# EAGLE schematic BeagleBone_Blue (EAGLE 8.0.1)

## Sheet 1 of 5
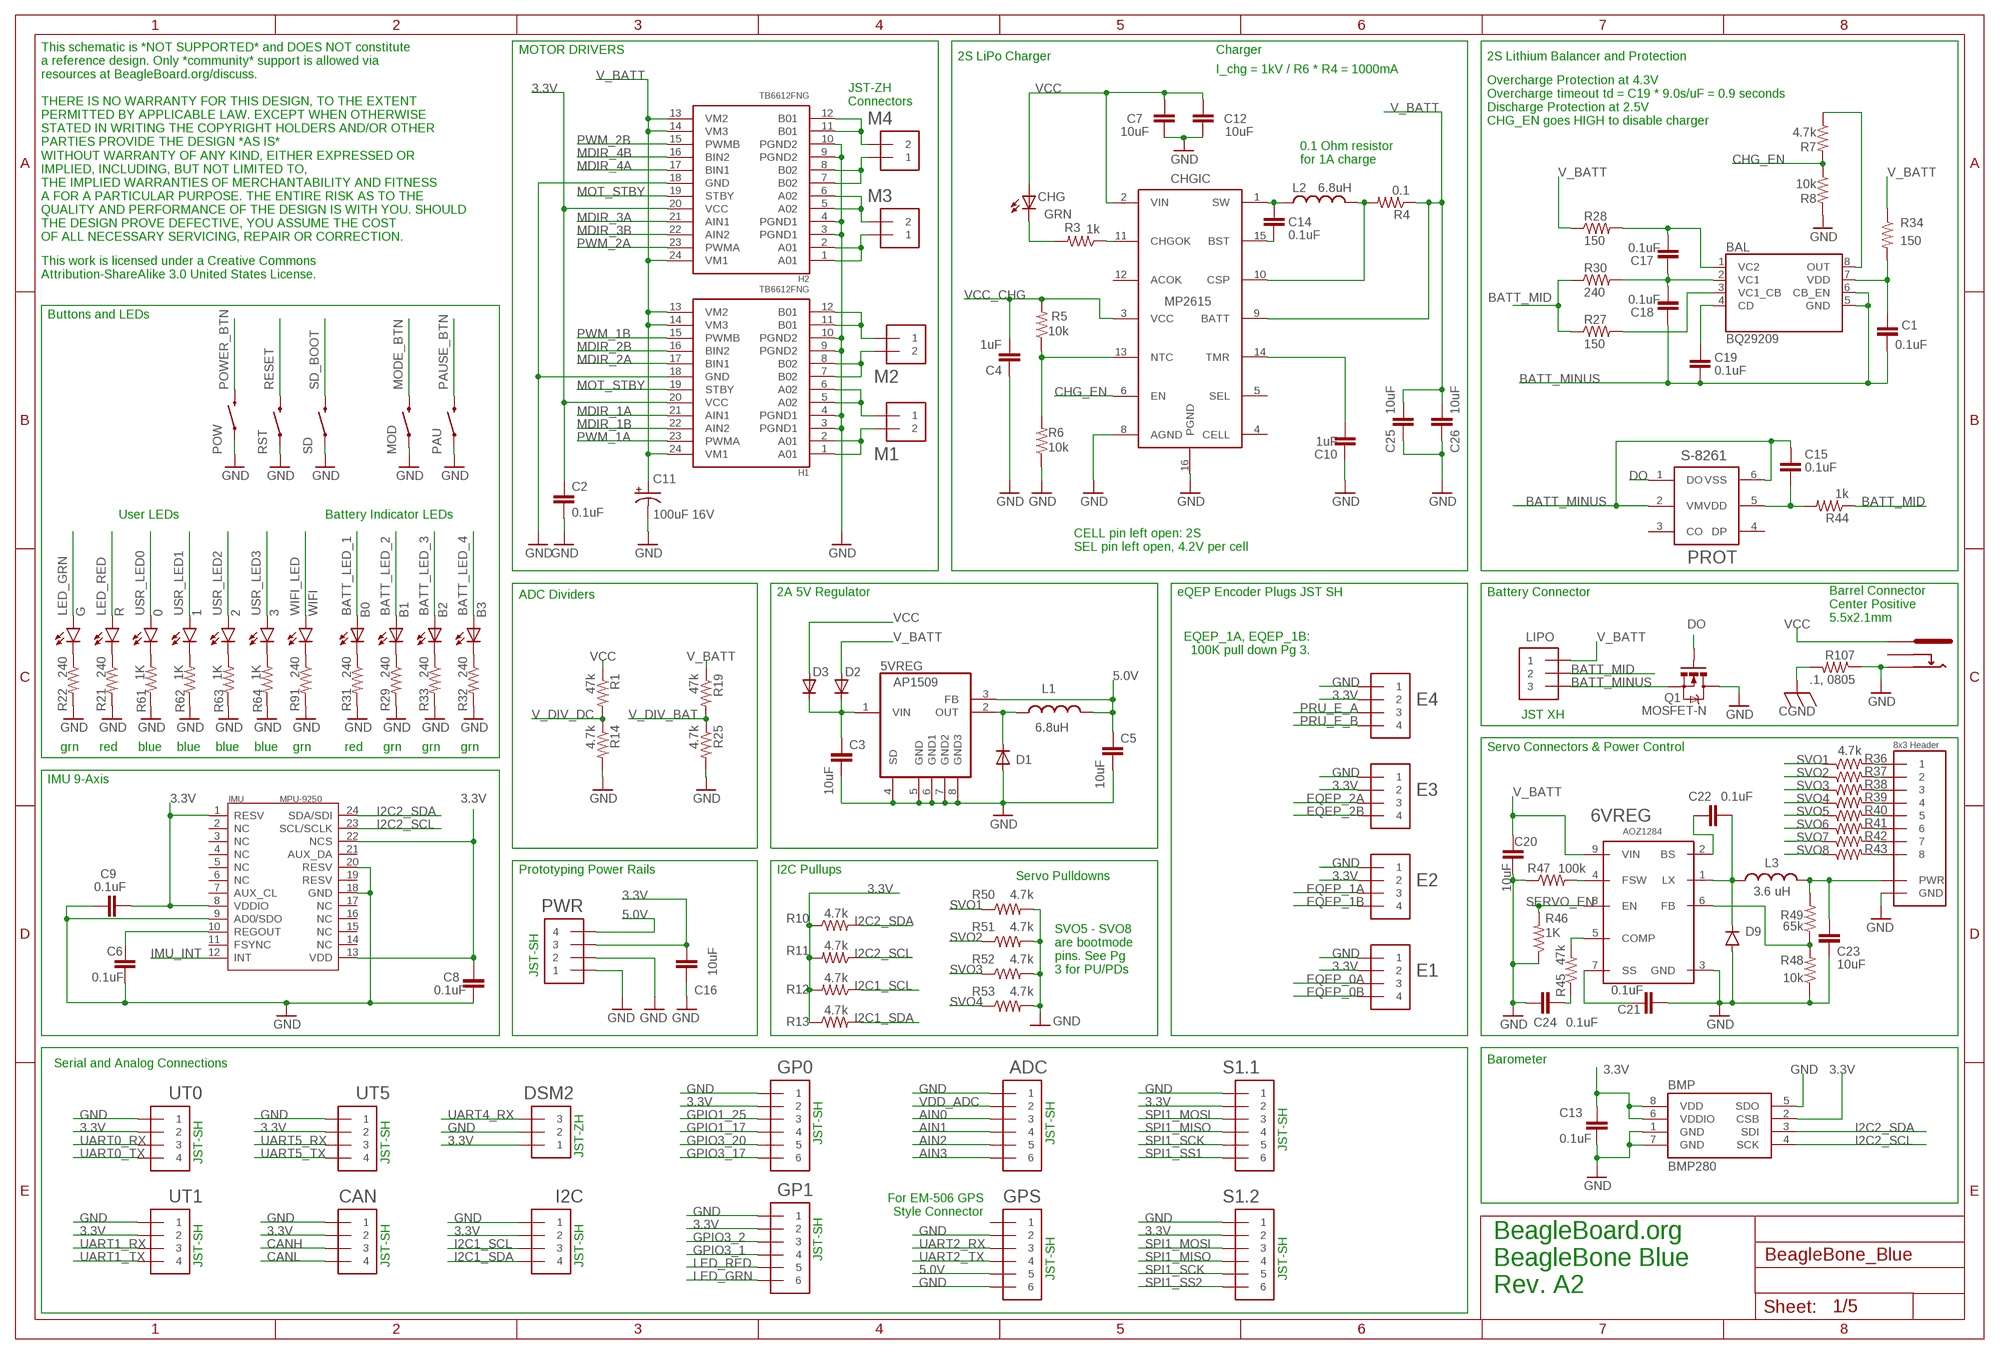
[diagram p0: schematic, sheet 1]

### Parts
0  BLUE  LED0603  [BEAGLEBONE_BLUE_LED-0603]
1  BLUE  LED0603  [BEAGLEBONE_BLUE_LED-0603]
2  BLUE  LED0603  [BEAGLEBONE_BLUE_LED-0603]
3  BLUE  LED0603  [BEAGLEBONE_BLUE_LED-0603]
5VREG  AP1509SOIC-8-TIGHT  [BEAGLEBONE_BLUE_SO08-TIGHT]
6VREG  AOZ1284  [SO08-EXPOSED]
12V  PJ-102B_POWER_CON  [PJ-102B_POWER_CON]
ADC  JST_SH_6  [JST_SH_6]
B0  RED  LED0603  [LED-0603]
B1  GREEN  LED0603  [LED-0603]
B2  GREEN  LED0603  [LED-0603]
B3  GREEN  LED0603  [LED-0603]
BAL  BQ29209  [8-SON_3X3MM]
BMP  BMP280  [BMP280]
C1  0.1uF  CAP0402-CAP  [0402-CAP]
C2  0.1uF  CAP0402-CAP  [0402-CAP]
C3  10uF  CAP0805  [0805]
C4  1uF  CAP0402-CAP  [0402-CAP]
C5  10uF  CAP0805  [0805]
C6  0.1uF  CAP0402-CAP  [0402-CAP]
C7  10uF  CAP0805  [0805]
C8  0.1uF  CAP0402-CAP  [0402-CAP]
C9  0.1uF  CAP0402-CAP  [0402-CAP]
C10  1uF  CAP0402-CAP  [0402-CAP]
C11  100uF 16V  CPOL-USD  [PANASONIC_D]
C12  10uF  CAP0805  [0805]
C13  0.1uF  CAP0402-CAP  [0402-CAP]
C14  0.1uF  CAP0402-CAP  [0402-CAP]
C15  0.1uF  CAP0402-CAP  [0402-CAP]
C16  10uF  CAP0805  [0805]
C17  0.1uF  CAP0402-CAP  [0402-CAP]
C18  0.1uF  CAP0402-CAP  [0402-CAP]
C19  0.1uF  CAP0402-CAP  [0402-CAP]
C20  10uF  CAP0805  [0805]
C21  0.1uF  CAP0402-CAP  [0402-CAP]
C22  0.1uF  CAP0402-CAP  [0402-CAP]
C23  10uF  CAP0805  [0805]
C24  0.1uF  CAP0402-CAP  [0402-CAP]
C25  10uF  CAP0805  [0805]
C26  10uF  CAP0805  [0805]
CAN  JST_SH_4  [JST_SH_4_SMD]
CHG  GRN  LED0603  [LED-0603]
CHGIC  MP2615  [MP2615]
D1  DIODE_SOD-123FL  [ADAFRUIT_SOD-123FL]
D2  DIODE_SOD-123FL  [ADAFRUIT_SOD-123FL]
D3  DIODE_SOD-123FL  [ADAFRUIT_SOD-123FL]
D9  DIODEDO214AA  [DO-214AA]
DSM2  JST_ZH_3  [JST_ZH_3]
E1  JST_SH_4  [JST_SH_4_SMD]
E2  JST_SH_4  [JST_SH_4_SMD]
E3  JST_SH_4  [JST_SH_4_SMD]
E4  JST_SH_4  [JST_SH_4_SMD]
G  GREEN  LED0603  [BEAGLEBONE_BLUE_LED-0603]
GP0  JST_SH_6  [JST_SH_6]
GP1  JST_SH_6  [JST_SH_6]
GPS  JST_SH_6  [JST_SH_6]
H1  TB6612FNG  [SSOP24]
H2  TB6612FNG  [SSOP24]
I2C  JST_SH_4  [JST_SH_4_SMD]
IMU  MPU-9250  [QFN24G-0.4-3X3MM]
J2  STRAWSON_EAGLE_LIB_SERVO_HEADERS_8X  [STRAWSON_EAGLE_LIB_3X8_0.1"_HEADER]
L1  6.8uH  INDUCTORBOURNS_SRN6045  [SRN6045]
L2  6.8uH  INDUCTORBOURNS_SRN6045  [SRN6045]
L3  3.6 uH  INDUCTOR  [8X8MM_INDUCTOR]
LIPO  BATTERY  JST_XH_3-PIN  [JST_XH_3-PIN]
M1  JST_ZH_2  [JST_ZH_2]
M2  JST_ZH_2  [JST_ZH_2]
M3  JST_ZH_2  [JST_ZH_2]
M4  JST_ZH_2  [JST_ZH_2]
MOD  SWITCH-MOMENTARY-2SMD-1101NE  [TACTILE-SWITCH-1101NE]
PAU  SWITCH-MOMENTARY-2SMD-1101NE  [TACTILE-SWITCH-1101NE]
POW  SWITCH-MOMENTARY-2SMD-1101NE  [TACTILE-SWITCH-1101NE]
PROT  S-8261  [SOT-236]
PWR  JST_SH_4  [JST_SH_4_SMD]
Q1  MOSFET-N  MOSFET-NCHANNEL  [SO08-TIGHT]
R  RED  LED0603  [BEAGLEBONE_BLUE_LED-0603]
R1  47k  RESISTOR0402-RES  [0402-RES]
R3  1k  RESISTOR0402-RES  [0402-RES]
R4  0.1  RESISTOR0603  [0603-RES]
R5  10k  RESISTOR0402-RES  [0402-RES]
R6  10k  RESISTOR0402-RES  [0402-RES]
R7  4.7k  RESISTOR0402-RES  [0402-RES]
R8  10k  RESISTOR0402-RES  [0402-RES]
R10  4.7k  RESISTOR0402-RES  [0402-RES]
R11  4.7k  RESISTOR0402-RES  [0402-RES]
R12  4.7k  RESISTOR0402-RES  [0402-RES]
R13  4.7k  RESISTOR0402-RES  [0402-RES]
R14  4.7k  RESISTOR0402-RES  [0402-RES]
R19  47k  RESISTOR0402-RES  [0402-RES]
R21  240  RESISTOR0402-RES  [0402-RES]
R22  240  RESISTOR0402-RES  [0402-RES]
R25  4.7k  RESISTOR0402-RES  [0402-RES]
R27  150  RESISTOR0402-RES  [0402-RES]
R28  150  RESISTOR0402-RES  [0402-RES]
R29  240  RESISTOR0402-RES  [0402-RES]
R30  240  RESISTOR0402-RES  [0402-RES]
R31  240  RESISTOR0402-RES  [0402-RES]
R32  240  RESISTOR0402-RES  [0402-RES]
R33  240  RESISTOR0402-RES  [0402-RES]
R34  150  RESISTOR0402-RES  [0402-RES]
R36  4.7k  RESISTOR0402-RES  [0402-RES]
R37  4.7k  RESISTOR0402-RES  [0402-RES]
R38  4.7k  RESISTOR0402-RES  [0402-RES]
R39  4.7k  RESISTOR0402-RES  [0402-RES]
R40  4.7k  RESISTOR0402-RES  [0402-RES]
R41  4.7k  RESISTOR0402-RES  [0402-RES]
R42  4.7k  RESISTOR0402-RES  [0402-RES]
R43  4.7k  RESISTOR0402-RES  [0402-RES]
R44  1k  RESISTOR0402-RES  [0402-RES]
R45  47k  RESISTOR0402-RES  [0402-RES]
R46  1K  RESISTOR0402-RES  [0402-RES]
R47  100k  RESISTOR0402-RES  [0402-RES]
R48  10k  RESISTOR0402-RES  [0402-RES]
R49  65k  RESISTOR0402-RES  [0402-RES]
R50  4.7k  RESISTOR0402-RES  [0402-RES]
R51  4.7k  RESISTOR0402-RES  [0402-RES]
R52  4.7k  RESISTOR0402-RES  [0402-RES]
R53  4.7k  RESISTOR0402-RES  [0402-RES]
R61  1K  RESISTOR0402-RES  [0402-RES]
R62  1K  RESISTOR0402-RES  [0402-RES]
R63  1K  RESISTOR0402-RES  [0402-RES]
R64  1K  RESISTOR0402-RES  [0402-RES]
R91  240  RESISTOR0402-RES  [0402-RES]
R107  .1, 0805  R-US_R0805  [R0805]
RST  SWITCH-MOMENTARY-2SMD-1101NE  [TACTILE-SWITCH-1101NE]
S1.1  JST_SH_6  [JST_SH_6]
S1.2  JST_SH_6  [JST_SH_6]
SD  SWITCH-MOMENTARY-2SMD-1101NE  [TACTILE-SWITCH-1101NE]
UT0  JST_SH_4  [JST_SH_4_SMD]
UT1  JST_SH_4  [JST_SH_4_SMD]
UT5  JST_SH_4  [JST_SH_4_SMD]
WIFI  GREEN  LED0603  [BEAGLEBONE_BLUE_LED-0603]

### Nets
3.3V: BMP.2(CSB) BMP.6(VDDIO) BMP.8(VDD) C2.2 C8.1 C9.2 C13.1 C16.1 CAN.2 DSM2.P$1 E1.2 E2.2 E3.2 E4.2 GP0.2 GP1.2 H1.20(VCC) H2.20(VCC) I2C.2 IMU.1(RESV) IMU.8(VDDIO) IMU.13(VDD) IMU.22(NCS) PWR.3 R10.1 R11.2 R12.2 R13.1 S1.1.2 S1.2.2 UT0.2 UT1.2 UT5.2 ; also sheet 2,3,5
5.0V [power]: 5VREG.3(FB) C5.1 GPS.5 L1.2 PWR.4 ; also sheet 2,3
AIN0: ADC.3 ; also sheet 3
AIN1: ADC.4 ; also sheet 3
AIN2: ADC.5 ; also sheet 3
AIN3: ADC.6 ; also sheet 3
BATT_LED_1: B0.A ; also sheet 2
BATT_LED_2: B1.A ; also sheet 3
BATT_LED_3: B2.A ; also sheet 2
BATT_LED_4: B3.A ; also sheet 2
BATT_MID: LIPO.P$2 R27.1 R30.1 R44.1
BATT_MINUS: BAL.5(GND) BAL.6(CB_EN) C1.2 C15.1 C18.1 C19.2 LIPO.P$3 PROT.2(VM) PROT.6(VSS) Q1.1(S) Q1.2(S) Q1.3(S)
CANH: CAN.3 ; also sheet 2
CANL: CAN.4 ; also sheet 2
CGND: R107.2 ; also sheet 2,3,4
CHG_EN: CHGIC.6(EN) R7.2 R8.1
CO: BAL.8(OUT) R7.1
DO: PROT.1(DO) Q1.4(G)
EQEP_0A: E1.3 ; also sheet 2
EQEP_0B: E1.4 ; also sheet 2
EQEP_1A: E2.3 ; also sheet 3
EQEP_1B: E2.4 ; also sheet 3
EQEP_2A: E3.3 ; also sheet 2
EQEP_2B: E3.4 ; also sheet 2
GND [ground]: 5VREG.4(SD) 5VREG.5(GND) 5VREG.6(GND1) 5VREG.7(GND2) 5VREG.8(GND3) 6VREG.3(GND) 12V.OUT ADC.1 BMP.1(GND) BMP.5(SDO) BMP.7(GND) C2.1 C3.2 C4.1 C5.2 C6.2 C7.2 C8.2 C9.1 C10.1 C11.- C12.2 C13.2 C16.2 C20.1 C21.1 C23.1 C24.1 C25.2 C26.2 CAN.1 CHGIC.8(AGND) CHGIC.16(PGND) D1.A D9.A DSM2.P$2 E1.1 E2.1 E3.1 E4.1 GP0.1 GP1.1 GPS.2 GPS.6 H1.3(PGND1) H1.4(PGND1) H1.9(PGND2) H1.10(PGND2) H1.18(GND) H2.3(PGND1) H2.4(PGND1) H2.9(PGND2) H2.10(PGND2) H2.18(GND) I2C.1 IMU.9(AD0/SDO) IMU.18(GND) IMU.20(RESV) J2.P$13(GND) J2.P$14(GND) J2.P$15(GND) J2.P$16(GND) J2.P$17(GND) J2.P$18(GND) J2.P$23(GND) J2.P$24(GND) MOD.1 PAU.1 POW.1 PWR.1 PWR.2 Q1.5(D) Q1.6(D) Q1.7(D) Q1.8(D) R6.1 R8.2 R14.2 R21.2 R22.2 R25.2 R29.2 R31.2 R32.2 R33.2 R46.1 R47.1 R48.1 R50.2 R51.2 R52.2 R53.2 R61.1 R62.1 R63.1 R64.1 R91.2 R107.1 RST.1 S1.1.1 S1.2.1 SD.1 UT0.1 UT1.1 UT5.1 ; also sheet 2,3,4,5
GPIO1_17: GP0.4 ; also sheet 2
GPIO1_25: GP0.3 ; also sheet 3
GPIO3_1: GP1.4 ; also sheet 3
GPIO3_2: GP1.3 ; also sheet 3
GPIO3_17: GP0.6 ; also sheet 2
GPIO3_20: GP0.5 ; also sheet 2
I2C1_SCL: I2C.3 R12.1 ; also sheet 2
I2C1_SDA: I2C.4 R13.2 ; also sheet 2
I2C2_SCL: BMP.4(SCK) IMU.23(SCL/SCLK) R11.1 ; also sheet 2
I2C2_SDA: BMP.3(SDI) IMU.24(SDA/SDI) R10.2 ; also sheet 2
IMU_INT: IMU.12(INT) ; also sheet 2
L3: B2.C R33.1
L4: B3.C R32.1
LED_GRN: G.A GP1.6 ; also sheet 2
LED_RED: GP1.5 R.A ; also sheet 2
MDIR_1A: H1.21(AIN1) ; also sheet 2
MDIR_1B: H1.22(AIN2) ; also sheet 2
MDIR_2A: H1.17(BIN1) ; also sheet 2
MDIR_2B: H1.16(BIN2) ; also sheet 3
MDIR_3A: H2.21(AIN1) ; also sheet 3
MDIR_3B: H2.22(AIN2) ; also sheet 3
MDIR_4A: H2.17(BIN1) ; also sheet 3
MDIR_4B: H2.16(BIN2) ; also sheet 3
MODE_BTN: MOD.2 ; also sheet 2
MOT1A: H1.1(A01) H1.2(A01) M1.P$2
MOT1B: H1.5(A02) H1.6(A02) M1.P$1
MOT2A: H1.11(B01) H1.12(B01) M2.P$1
MOT2B: H1.7(B02) H1.8(B02) M2.P$2
MOT3A: H2.1(A01) H2.2(A01) M3.P$1
MOT3B: H2.5(A02) H2.6(A02) M3.P$2
MOT4A: H2.11(B01) H2.12(B01) M4.P$2
MOT4B: H2.7(B02) H2.8(B02) M4.P$1
MOT_STBY: H1.19(STBY) H2.19(STBY) ; also sheet 2
N$1: J2.P$1 R36.2
N$3: G.C R22.1
N$4: BAL.2(VC1) C17.1 C18.2 R30.2
N$6: R21.1 R.C
N$8: BAL.1(VC2) C17.2 R28.2
N$10: 6VREG.7(SS) C21.2
N$11: C15.2 PROT.5(VDD) R44.2
N$14: C6.1 IMU.10(REGOUT)
N$15: C14.1 CHGIC.15(BST)
N$16: 5VREG.2(OUT) D1.C L1.1
N$17: CHG.C R3.2
N$18: CHGIC.11(CHGOK) R3.1
N$20: R91.1 WIFI.C
N$24: BAL.4(CD) C19.1
N$25: J2.P$2 R37.2
N$29: BAL.7(VDD) C1.1 R34.2
N$30: J2.P$3 R38.2
N$38: J2.P$4 R39.2
N$47: 0.C R61.2
N$48: B1.C R29.1
N$49: B0.C R31.1
N$50: BAL.3(VC1_CB) R27.2
N$51: J2.P$5 R40.2
N$52: J2.P$6 R41.2
N$53: 6VREG.2(BS) C22.1
N$54: J2.P$19 R42.2
N$55: C14.2 CHGIC.1(SW) L2.1
N$56: J2.P$20 R43.2
N$57: 1.C R62.2
N$58: 2.C R63.2
N$59: 3.C R64.2
N$60: 6VREG.1(LX) C22.2 D9.C L3.1
N$61: 6VREG.4(FSW) R47.2
N$62: C23.2 J2.P$7(PWR) J2.P$8(PWR) J2.P$9(PWR) J2.P$10(PWR) J2.P$11(PWR) J2.P$12(PWR) J2.P$21(PWR) J2.P$22(PWR) L3.2 R49.2
N$63: 6VREG.5(COMP) R45.2
N$65: 6VREG.6(FB) R48.2 R49.1
N$66: C24.2 R45.1
N$67: CHGIC.10(CSP) L2.2 R4.2
N$69: C10.2 CHGIC.14(TMR)
N$71: CHGIC.13(NTC) R5.1 R6.2
N$79: 5VREG.1(VIN) C3.1 D2.C D3.C
PAUSE_BTN: PAU.2 ; also sheet 2
POWER_BTN: POW.2 ; also sheet 2
PRU_E_A: E4.3 ; also sheet 2
PRU_E_B: E4.4 ; also sheet 2
PWM_1A: H1.23(PWMA) ; also sheet 2
PWM_1B: H1.15(PWMB) ; also sheet 2
PWM_2A: H2.23(PWMA) ; also sheet 2
PWM_2B: H2.15(PWMB) ; also sheet 2
RESET: RST.2 ; also sheet 2
SD_BOOT: SD.2 ; also sheet 3
SERVO_EN: 6VREG.8(EN) R46.2 ; also sheet 3
SPI1_MISO: S1.1.4 S1.2.4 ; also sheet 2
SPI1_MOSI: S1.1.3 S1.2.3 ; also sheet 2
SPI1_SCK: S1.1.5 S1.2.5 ; also sheet 2
SPI1_SS1: S1.1.6 ; also sheet 3
SPI1_SS2: S1.2.6 ; also sheet 2
SVO1: R36.1 R50.1 ; also sheet 3
SVO2: R37.1 R51.1 ; also sheet 3
SVO3: R38.1 R52.1 ; also sheet 3
SVO4: R39.1 R53.1 ; also sheet 3
SVO5: R40.1 ; also sheet 3
SVO6: R41.1 ; also sheet 3
SVO7: R42.1 ; also sheet 3
SVO8: R43.1 ; also sheet 3
UART0_RX: UT0.3 ; also sheet 2
UART0_TX: UT0.4 ; also sheet 2
UART1_RX: UT1.3 ; also sheet 2
UART1_TX: UT1.4 ; also sheet 2
UART2_RX: GPS.3 ; also sheet 2
UART2_TX: GPS.4 ; also sheet 2
UART4_RX: DSM2.P$3 ; also sheet 2
UART5_RX: UT5.3 ; also sheet 3
UART5_TX: UT5.4 ; also sheet 3
USR_LED0: 0.A ; also sheet 2
USR_LED1: 1.A ; also sheet 2
USR_LED2: 2.A ; also sheet 2
USR_LED3: 3.A ; also sheet 2
V_BATT: 6VREG.9(VIN) C11.+ C20.2 C25.1 C26.1 CHGIC.9(BATT) D2.A H1.13(VM2) H1.14(VM3) H1.24(VM1) H2.13(VM2) H2.14(VM3) H2.24(VM1) LIPO.P$1 R4.1 R19.1 R28.1 R34.1
V_DIV_BAT: R19.2 R25.1 ; also sheet 3
V_DIV_DC: R1.2 R14.1 ; also sheet 3
VCC: 12V.IN C7.1 C12.1 CHG.A CHGIC.2(VIN) D3.A R1.1
VCC_CHG: C4.2 CHGIC.3(VCC) R5.2
VDD_ADC: ADC.2 ; also sheet 3,4
WIFI_LED: WIFI.A ; also sheet 2
Unconnected: 12V.OUT_CON CHGIC.4(CELL) CHGIC.5(SEL) CHGIC.12(ACOK) GPS.1 IMU.2(NC) IMU.3(NC) IMU.4(NC) IMU.5(NC) IMU.6(NC) IMU.7(AUX_CL) IMU.11(FSYNC) IMU.14(NC) IMU.15(NC) IMU.16(NC) IMU.17(NC) IMU.19(RESV) IMU.21(AUX_DA) PROT.3(CO) PROT.4(DP)

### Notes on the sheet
- MOTOR DRIVERS | Charger
- 2S LiPo Charger | 2S Lithium Balancer and Protection
- I_chg = 1kV / R6 * R4 = 1000mA
- JST-ZH
  Connectors
- Overcharge Protection at 4.3V
  Overcharge timeout td = C19 * 9.0s/uF = 0.9 seconds
  Discharge Protection at 2.5V
  CHG_EN goes HIGH to disable charger
- 0.1 Ohm resistor
  for 1A charge
- This schematic is *NOT SUPPORTED* and DOES NOT constitute 
  a reference design. Only *community* support is allowed via 
  resources at BeagleBoard.org/discuss. 
  
  THERE IS NO WARRANTY FOR THIS DESIGN, TO THE EXTENT 
  PERMITTED BY APPLICABLE LAW. EXCEPT WHEN OTHERWISE 
  STATED IN WRITING THE COPYRIGHT HOLDERS AND/OR OTHER 
  PARTIES PROVIDE THE DESIGN *AS IS*
  WITHOUT WARRANTY OF ANY KIND, EITHER EXPRESSED OR 
  IMPLIED, INCLUDING, BUT NOT LIMITED TO, 
  THE IMPLIED WARRANTIES OF MERCHANTABILITY AND FITNESS 
  A FOR A PARTICULAR PURPOSE. THE ENTIRE RISK AS TO THE 
  QUALITY AND PERFORMANCE OF THE DESIGN IS WITH YOU. SHOULD 
  THE DESIGN PROVE DEFECTIVE, YOU ASSUME THE COST 
  OF ALL NECESSARY SERVICING, REPAIR OR CORRECTION.
- This work is licensed under a Creative Commons 
  Attribution-ShareAlike 3.0 United States License.
- Buttons and LEDs
- User LEDs | Battery Indicator LEDs
- CELL pin left open: 2S
  SEL pin left open, 4.2V per cell
- ADC Dividers
- 2A 5V Regulator | eQEP Encoder Plugs JST SH | Battery Connector
- Barrel Connector
  Center Positive
  5.5x2.1mm
- EQEP_1A, EQEP_1B: 
    100K pull down Pg 3.
- JST XH
- grn | red | blue | blue | blue | blue | grn | red | grn | grn | grn | Servo Connectors & Power Control
- IMU 9-Axis
- Prototyping Power Rails | I2C Pullups
- Servo Pulldowns
- SVO5 - SVO8 
  are bootmode 
  pins. See Pg 
  3 for PU/PDs
- JST-SH
- Barometer
- Serial and Analog Connections
- JST-SH | JST-SH
- JST-SH
- JST-ZH
- JST-SH | JST-SH
- For EM-506 GPS
  Style Connector
- JST-SH
- JST-SH | JST-SH | JST-SH
- JST-SH | JST-SH
- BeagleBoard.org
  BeagleBone Blue
  Rev. A2

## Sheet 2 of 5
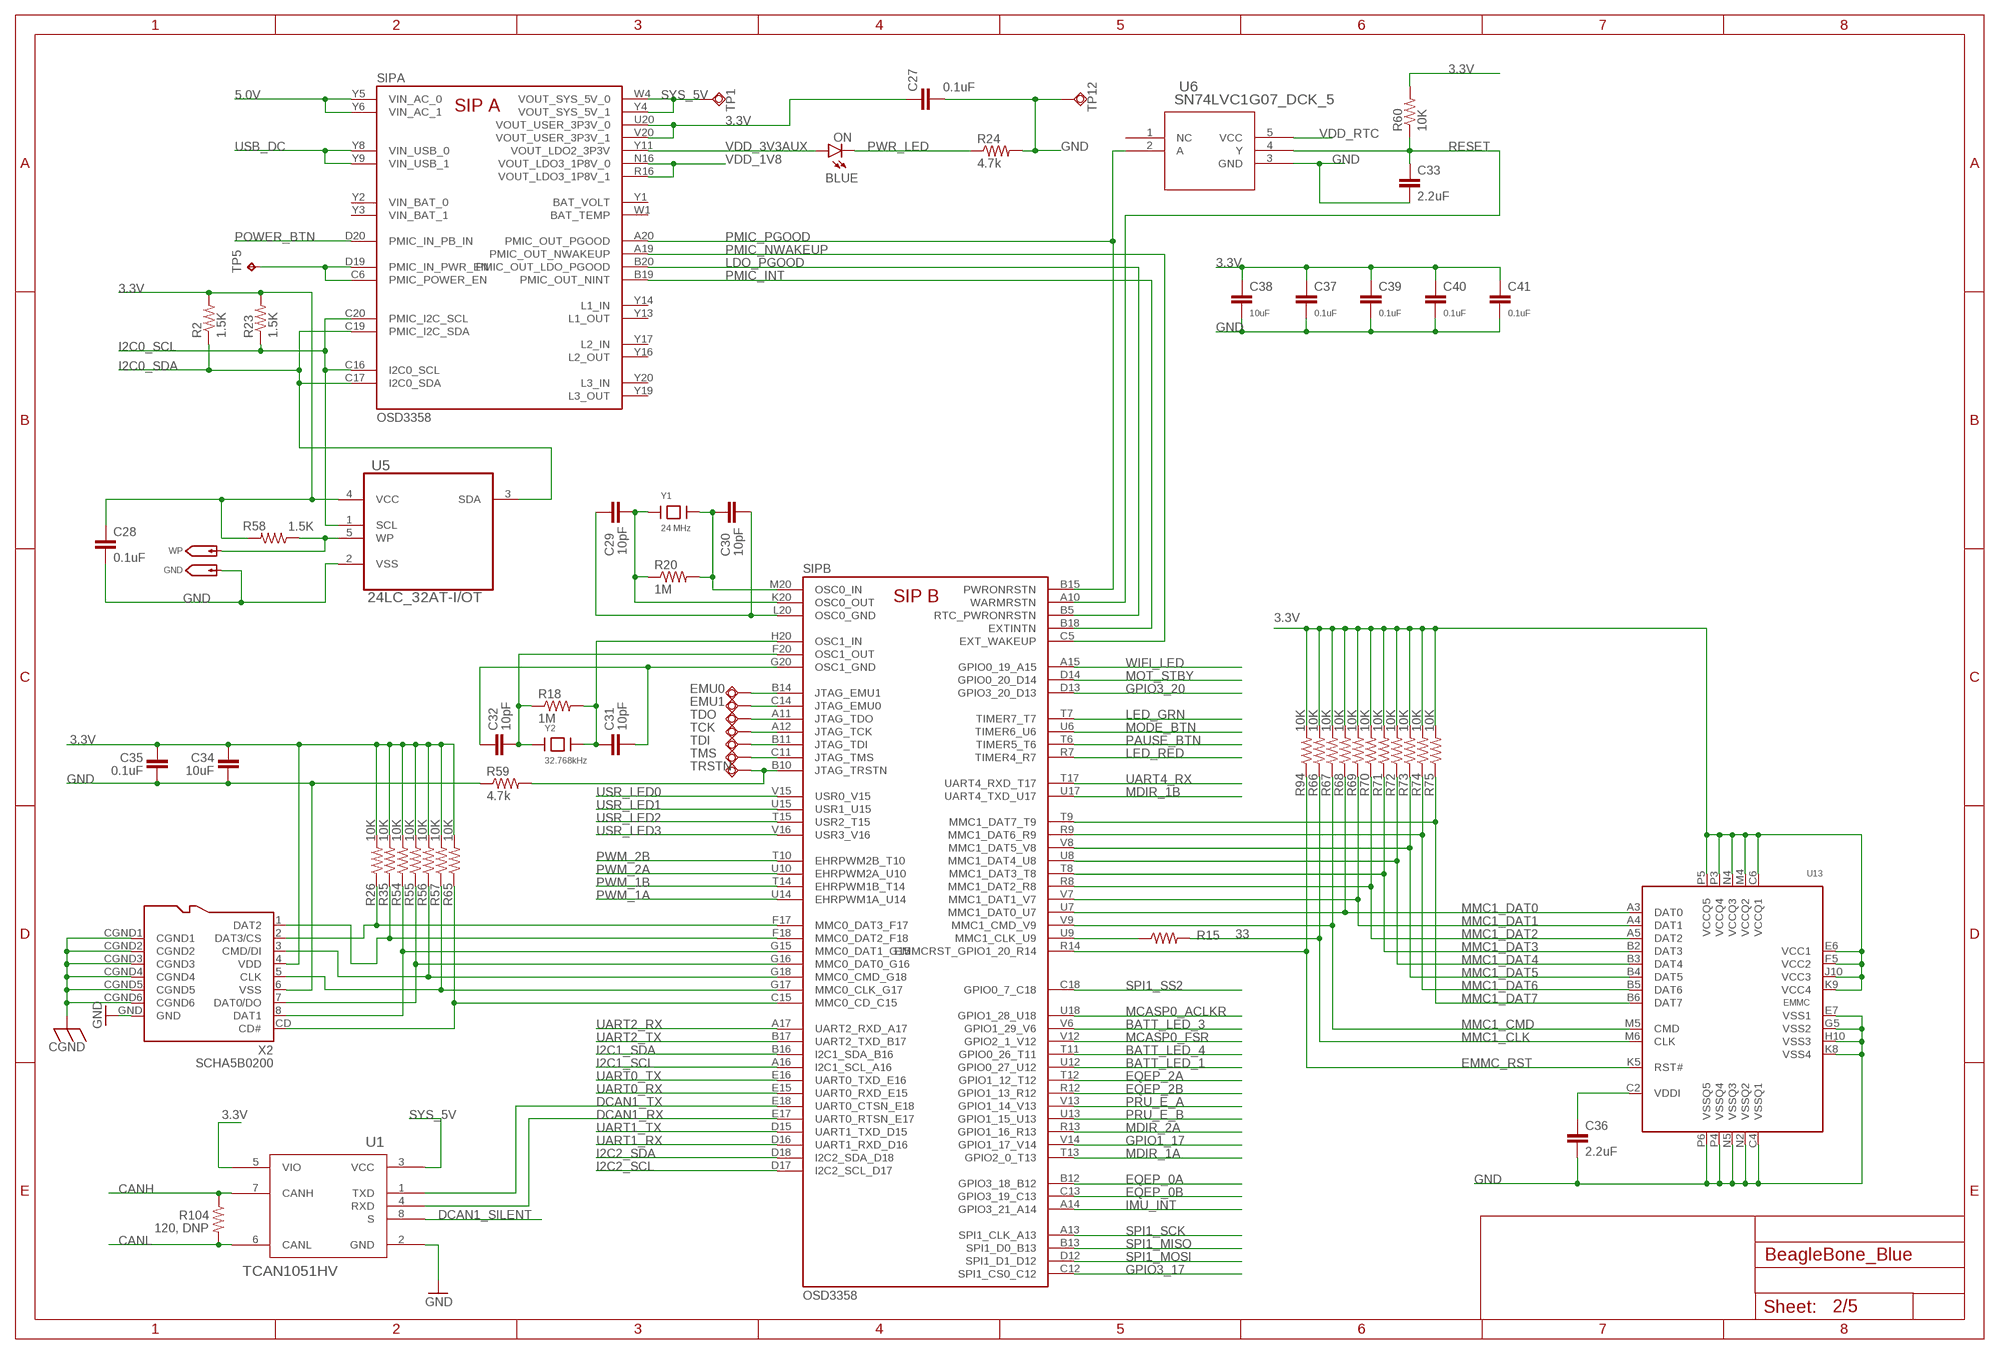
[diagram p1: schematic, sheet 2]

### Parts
C27  0.1uF  CAP0402-CAP  [0402-CAP]
C28  0.1uF  CAP0402-CAP  [0402-CAP]
C29  10pF  CAP0402-CAP  [0402-CAP]
C30  10pF  CAP0402-CAP  [0402-CAP]
C31  10pF  CAP0402-CAP  [0402-CAP]
C32  10pF  CAP0402-CAP  [0402-CAP]
C33  2.2uF  CAP0402-CAP  [0402-CAP]
C34  10uF  CAP0805  [0805]
C35  0.1uF  CAP0402-CAP  [0402-CAP]
C36  2.2uF  CAP0402-CAP  [0402-CAP]
C37  0.1uF  CAP0402-CAP  [0402-CAP]
C38  10uF  CAP0805  [0805]
C39  0.1uF  CAP0402-CAP  [0402-CAP]
C40  0.1uF  CAP0402-CAP  [0402-CAP]
C41  0.1uF  CAP0402-CAP  [0402-CAP]
EMU0  TPSQB1,27  [B1,27]
EMU1  TPSQB1,27  [B1,27]
GND  GHI2_TESTPAD/W_HOLE_1X1  [GHI2_TESTPAD/W_HOLE_1X1]
ON  BLUE  LED0603  [BEAGLEBONE_BLUE_LED-0603]
R2  1.5K  RESISTOR0402-RES  [0402-RES]
R15  33  RESISTOR0402-RES  [0402-RES]
R18  1M  RESISTOR0402-RES  [0402-RES]
R20  1M  RESISTOR0402-RES  [0402-RES]
R23  1.5K  RESISTOR0402-RES  [0402-RES]
R24  4.7k  RESISTOR0402-RES  [0402-RES]
R26  10K  RESISTOR0402-RES  [0402-RES]
R35  10K  RESISTOR0402-RES  [0402-RES]
R54  10K  RESISTOR0402-RES  [0402-RES]
R55  10K  RESISTOR0402-RES  [0402-RES]
R56  10K  RESISTOR0402-RES  [0402-RES]
R57  10K  RESISTOR0402-RES  [0402-RES]
R58  1.5K  RESISTOR0402-RES  [0402-RES]
R59  4.7k  RESISTOR0402-RES  [0402-RES]
R60  10K  RESISTOR0402-RES  [0402-RES]
R65  10K  RESISTOR0402-RES  [0402-RES]
R66  10K  RESISTOR0402-RES  [0402-RES]
R67  10K  RESISTOR0402-RES  [0402-RES]
R68  10K  RESISTOR0402-RES  [0402-RES]
R69  10K  RESISTOR0402-RES  [0402-RES]
R70  10K  RESISTOR0402-RES  [0402-RES]
R71  10K  RESISTOR0402-RES  [0402-RES]
R72  10K  RESISTOR0402-RES  [0402-RES]
R73  10K  RESISTOR0402-RES  [0402-RES]
R74  10K  RESISTOR0402-RES  [0402-RES]
R75  10K  RESISTOR0402-RES  [0402-RES]
R94  10K  RESISTOR0402-RES  [0402-RES]
R104  120, DNP  RESISTOR0603  [0603-RES]
SIP  OSD3358  [BEAGLEBONE_BLUE_OSD3358]
TCK  TPSQB1,27  [B1,27]
TDI  TPSQB1,27  [B1,27]
TDO  TPSQB1,27  [B1,27]
TMS  TPSQB1,27  [B1,27]
TP1  TPSQB1,27  [B1,27]
TP5  TPB0,65  [BEAGLEBONE_BLUE_B0,65]
TP12  TPSQB1,27  [B1,27]
TRSTN  TPSQB1,27  [B1,27]
U1  TCAN1051HV  [BEAGLEBONE_BLUE_D8]
U5  24LC_32AT-I/OT  [SOT95P290X145-5N]
U6  SN74LVC1G07_DCK_5  [BEAGLEBONE_BLUE_DCK5]
U13  EMMC  EMMC04G-S100-B08U  [MICRON_EMMC_153]
WP  GHI2_TESTPAD/W_HOLE_1X1  [GHI2_TESTPAD/W_HOLE_1X1]
X2  SCHA5B0200  SCHA5B0200(ALPS_USD)  [SCHA5B0200]
Y1  24 MHz  CRYSTAL_5X3.2MM  [CRYSTAL_5X3.2MM]
Y2  32.768kHz  CRYSTAL_3.2X1.5  [CRYSTAL_3.2X1.5]

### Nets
3.3V: C27.1 C28.1 C34.2 C35.2 C37.1 C38.1 C39.1 C40.1 C41.1 R2.2 R23.2 R26.2 R35.2 R54.2 R55.2 R56.2 R57.2 R58.2 R60.2 R65.2 R66.2 R67.2 R68.2 R69.2 R70.2 R71.2 R72.2 R73.2 R74.2 R75.2 R94.2 SIP.U20(A:VOUT_USER_3P3V_0) SIP.V20(A:VOUT_USER_3P3V_1) U1.5(VIO) U5.4(VCC) U13.C6(VCCQ1) U13.E6(VCC1) U13.F5(VCC2) U13.J10(VCC3) U13.K9(VCC4) U13.M4(VCCQ2) U13.N4(VCCQ3) U13.P3(VCCQ4) U13.P5(VCCQ5) X2.4(VDD) ; also sheet 1,3,5
5.0V [power]: SIP.Y5(A:VIN_AC_0) SIP.Y6(A:VIN_AC_1) ; also sheet 1,3
BATT_LED_1: SIP.U12(B:GPIO0_27_U12) ; also sheet 1
BATT_LED_3: SIP.V6(B:GPIO1_29_V6) ; also sheet 1
BATT_LED_4: SIP.T11(B:GPIO0_26_T11) ; also sheet 1
CANH: R104.1 U1.7(CANH) ; also sheet 1
CANL: R104.2 U1.6(CANL) ; also sheet 1
CGND: X2.CGND1 X2.CGND2 X2.CGND3 X2.CGND4 X2.CGND5 X2.CGND6 ; also sheet 1,3,4
DCAN1_RX: SIP.E17(B:UART0_RTSN_E17) U1.4(RXD)
DCAN1_SILENT: U1.8(S) ; also sheet 3
DCAN1_TX: SIP.E18(B:UART0_CTSN_E18) U1.1(TXD)
EMMC_RST: R94.1 SIP.R14(B:EMMCRST_GPIO1_20_R14) U13.K5(RST#)
EQEP_0A: SIP.B12(B:GPIO3_18_B12) ; also sheet 1
EQEP_0B: SIP.C13(B:GPIO3_19_C13) ; also sheet 1
EQEP_2A: SIP.T12(B:GPIO1_12_T12) ; also sheet 1
EQEP_2B: SIP.R12(B:GPIO1_13_R12) ; also sheet 1
GND [ground]: C27.2 C28.2 C33.2 C34.1 C35.1 C36.2 C37.2 C38.2 C39.2 C40.2 C41.2 GND.P$1(TP) R24.2 R59.1 TP12.TP U1.2(GND) U5.2(VSS) U6.3(GND) U13.C4(VSSQ1) U13.E7(VSS1) U13.G5(VSS2) U13.H10(VSS3) U13.K8(VSS4) U13.N2(VSSQ2) U13.N5(VSSQ3) U13.P4(VSSQ4) U13.P6(VSSQ5) X2.6(VSS) X2.GND ; also sheet 1,3,4,5
GPIO1_17: SIP.V14(B:GPIO1_17_V14) ; also sheet 1
GPIO3_17: SIP.C12(B:SPI1_CS0_C12) ; also sheet 1
GPIO3_20: SIP.D13(B:GPIO3_20_D13) ; also sheet 1
I2C0_SCL: R23.1 SIP.C16(A:I2C0_SCL) SIP.C20(A:PMIC_I2C_SCL) U5.1(SCL)
I2C0_SDA: R2.1 SIP.C17(A:I2C0_SDA) SIP.C19(A:PMIC_I2C_SDA) U5.3(SDA)
I2C1_SCL: SIP.A16(B:I2C1_SCL_A16) ; also sheet 1
I2C1_SDA: SIP.B16(B:I2C1_SDA_B16) ; also sheet 1
I2C2_SCL: SIP.D17(B:I2C2_SCL_D17) ; also sheet 1
I2C2_SDA: SIP.D18(B:I2C2_SDA_D18) ; also sheet 1
IMU_INT: SIP.A14(B:GPIO3_21_A14) ; also sheet 1
LDO_PGOOD: SIP.B5(B:RTC_PWRONRSTN) SIP.B20(A:PMIC_OUT_LDO_PGOOD)
LED_GRN: SIP.T7(B:TIMER7_T7) ; also sheet 1
LED_RED: SIP.R7(B:TIMER4_R7) ; also sheet 1
MCASP0_ACLKR: SIP.U18(B:GPIO1_28_U18) ; also sheet 5
MCASP0_FSR: SIP.V12(B:GPIO2_1_V12) ; also sheet 5
MDIR_1A: SIP.T13(B:GPIO2_0_T13) ; also sheet 1
MDIR_1B: SIP.U17(B:UART4_TXD_U17) ; also sheet 1
MDIR_2A: SIP.R13(B:GPIO1_16_R13) ; also sheet 1
MMC1_CLK: R15.2 R66.1 U13.M6(CLK)
MMC1_CMD: R67.1 SIP.V9(B:MMC1_CMD_V9) U13.M5(CMD)
MMC1_DAT0: R68.1 SIP.U7(B:MMC1_DAT0_U7) U13.A3(DAT0)
MMC1_DAT1: R69.1 SIP.V7(B:MMC1_DAT1_V7) U13.A4(DAT1)
MMC1_DAT2: R70.1 SIP.R8(B:MMC1_DAT2_R8) U13.A5(DAT2)
MMC1_DAT3: R71.1 SIP.T8(B:MMC1_DAT3_T8) U13.B2(DAT3)
MMC1_DAT4: R72.1 SIP.U8(B:MMC1_DAT4_U8) U13.B3(DAT4)
MMC1_DAT5: R73.1 SIP.V8(B:MMC1_DAT5_V8) U13.B4(DAT5)
MMC1_DAT6: R74.1 SIP.R9(B:MMC1_DAT6_R9) U13.B5(DAT6)
MMC1_DAT7: R75.1 SIP.T9(B:MMC1_DAT7_T9) U13.B6(DAT7)
MODE_BTN: SIP.U6(B:TIMER6_U6) ; also sheet 1
MOT_STBY: SIP.D14(B:GPIO0_20_D14) ; also sheet 1
N$2: R57.1 SIP.G17(B:MMC0_CLK_G17) X2.5(CLK)
N$5: R26.1 SIP.F17(B:MMC0_DAT3_F17) X2.2(DAT3/CS)
N$12: SIP.C6(A:PMIC_POWER_EN) SIP.D19(A:PMIC_IN_PWR_EN) TP5.TP
N$26: C30.1 R20.2 SIP.M20(B:OSC0_IN) Y1.2
N$27: C29.1 R20.1 SIP.K20(B:OSC0_OUT) Y1.1
N$28: R58.1 U5.5(WP) WP.P$1(TP)
N$31: C29.2 C30.2 SIP.L20(B:OSC0_GND)
N$32: C31.1 R18.2 SIP.H20(B:OSC1_IN) Y2.P$2
N$33: C32.2 R18.1 SIP.F20(B:OSC1_OUT) Y2.P$1
N$34: C31.2 C32.1 SIP.G20(B:OSC1_GND)
N$35: EMU0.TP SIP.B14(B:JTAG_EMU1)
N$36: EMU1.TP SIP.C14(B:JTAG_EMU0)
N$37: SIP.A11(B:JTAG_TDO) TDO.TP
N$39: SIP.A12(B:JTAG_TCK) TCK.TP
N$40: SIP.B11(B:JTAG_TDI) TDI.TP
N$41: SIP.C11(B:JTAG_TMS) TMS.TP
N$42: R59.2 SIP.B10(B:JTAG_TRSTN) TRSTN.TP
N$70: R54.1 SIP.G15(B:MMC0_DAT1_G15) X2.8(DAT1)
N$74: R56.1 SIP.G18(B:MMC0_CMD_G18) X2.3(CMD/DI)
N$75: R65.1 SIP.C15(B:MMC0_CD_C15) X2.CD(CD#)
N$77: R55.1 SIP.G16(B:MMC0_DAT0_G16) X2.7(DAT0/DO)
N$81: C36.1 U13.C2(VDDI)
N$85: R15.1 SIP.U9(B:MMC1_CLK_U9)
NTE: R35.1 SIP.F18(B:MMC0_DAT2_F18) X2.1(DAT2)
PAUSE_BTN: SIP.T6(B:TIMER5_T6) ; also sheet 1
PMIC_INT: SIP.B18(B:EXTINTN) SIP.B19(A:PMIC_OUT_NINT)
PMIC_NWAKEUP: SIP.A19(A:PMIC_OUT_NWAKEUP) SIP.C5(B:EXT_WAKEUP)
PMIC_PGOOD: SIP.A20(A:PMIC_OUT_PGOOD) SIP.B15(B:PWRONRSTN) U6.2(A)
POWER_BTN: SIP.D20(A:PMIC_IN_PB_IN) ; also sheet 1
PRU_E_A: SIP.V13(B:GPIO1_14_V13) ; also sheet 1
PRU_E_B: SIP.U13(B:GPIO1_15_U13) ; also sheet 1
PWM_1A: SIP.U14(B:EHRPWM1A_U14) ; also sheet 1
PWM_1B: SIP.T14(B:EHRPWM1B_T14) ; also sheet 1
PWM_2A: SIP.U10(B:EHRPWM2A_U10) ; also sheet 1
PWM_2B: SIP.T10(B:EHRPWM2B_T10) ; also sheet 1
PWR_LED: ON.C R24.1
RESET: C33.1 R60.1 SIP.A10(B:WARMRSTN) U6.4(Y) ; also sheet 1
SPI1_MISO: SIP.B13(B:SPI1_D0_B13) ; also sheet 1
SPI1_MOSI: SIP.D12(B:SPI1_D1_D12) ; also sheet 1
SPI1_SCK: SIP.A13(B:SPI1_CLK_A13) ; also sheet 1
SPI1_SS2: SIP.C18(B:GPIO0_7_C18) ; also sheet 1
SYS_5V [power]: SIP.W4(A:VOUT_SYS_5V_0) SIP.Y4(A:VOUT_SYS_5V_1) TP1.TP U1.3(VCC) ; also sheet 3
UART0_RX: SIP.E15(B:UART0_RXD_E15) ; also sheet 1
UART0_TX: SIP.E16(B:UART0_TXD_E16) ; also sheet 1
UART1_RX: SIP.D16(B:UART1_RXD_D16) ; also sheet 1
UART1_TX: SIP.D15(B:UART1_TXD_D15) ; also sheet 1
UART2_RX: SIP.A17(B:UART2_RXD_A17) ; also sheet 1
UART2_TX: SIP.B17(B:UART2_TXD_B17) ; also sheet 1
UART4_RX: SIP.T17(B:UART4_RXD_T17) ; also sheet 1
USB_DC [power]: SIP.Y8(A:VIN_USB_0) SIP.Y9(A:VIN_USB_1) ; also sheet 3
USR_LED0: SIP.V15(B:USR0_V15) ; also sheet 1
USR_LED1: SIP.U15(B:USR1_U15) ; also sheet 1
USR_LED2: SIP.T15(B:USR2_T15) ; also sheet 1
USR_LED3: SIP.V16(B:USR3_V16) ; also sheet 1
VDD_1V8: SIP.N16(A:VOUT_LDO3_1P8V_0) SIP.R16(A:VOUT_LDO3_1P8V_1) ; also sheet 4,5
VDD_3V3AUX: ON.A SIP.Y11(A:VOUT_LDO2_3P3V)
VDD_RTC: U6.5(VCC) ; also sheet 4
WIFI_LED: SIP.A15(B:GPIO0_19_A15) ; also sheet 1
Unconnected: SIP.W1(A:BAT_TEMP) SIP.Y1(A:BAT_VOLT) SIP.Y13(A:L1_OUT) SIP.Y14(A:L1_IN) SIP.Y16(A:L2_OUT) SIP.Y17(A:L2_IN) SIP.Y19(A:L3_OUT) SIP.Y20(A:L3_IN) U6.1(NC)

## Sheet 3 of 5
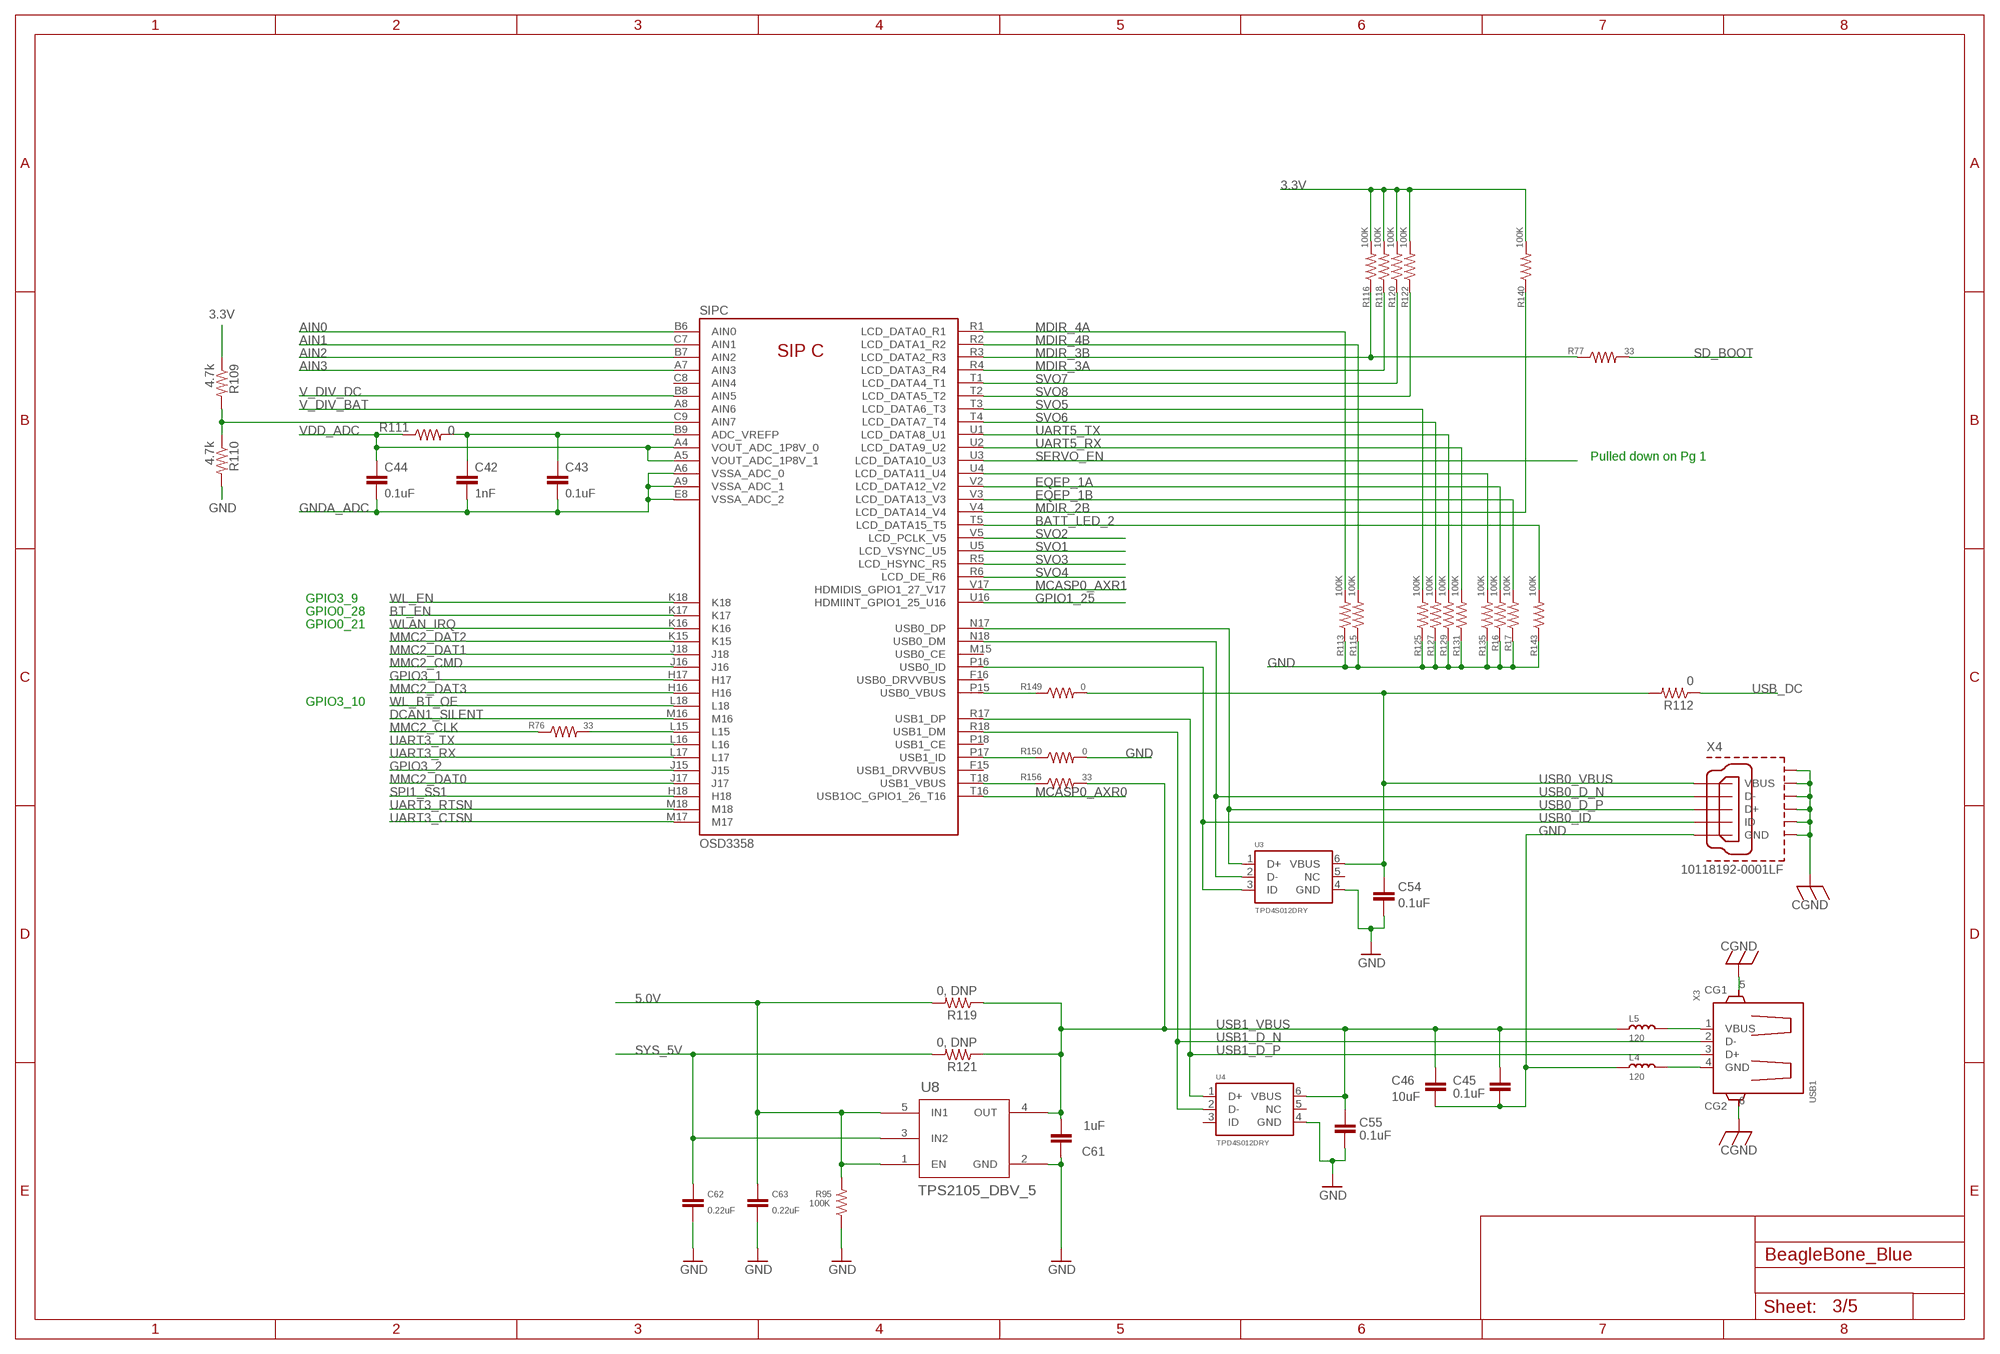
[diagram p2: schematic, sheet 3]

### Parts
C42  1nF  CAP0402-CAP  [0402-CAP]
C43  0.1uF  CAP0402-CAP  [0402-CAP]
C44  0.1uF  CAP0402-CAP  [0402-CAP]
C45  0.1uF  CAP0402-CAP  [0402-CAP]
C46  10uF  CAP0805  [0805]
C54  0.1uF  CAP0402-CAP  [0402-CAP]
C55  0.1uF  CAP0402-CAP  [0402-CAP]
C61  1uF  CAP0402-CAP  [0402-CAP]
C62  0.22uF  CAP0402-CAP  [0402-CAP]
C63  0.22uF  CAP0402-CAP  [0402-CAP]
L4  120  INDUCTOR/FERRITE-BEAD'0603'  [L0603]
L5  120  INDUCTOR/FERRITE-BEAD'0603'  [L0603]
R16  100K  RESISTOR0402-RES  [0402-RES]
R17  100K  RESISTOR0402-RES  [0402-RES]
R76  33  RESISTOR0402-RES  [0402-RES]
R77  33  RESISTOR0402-RES  [0402-RES]
R95  100K  RESISTOR0402-RES  [0402-RES]
R109  4.7k  RESISTOR0402-RES  [0402-RES]
R110  4.7k  RESISTOR0402-RES  [0402-RES]
R111  0  RESISTOR0402-RES  [0402-RES]
R112  0  RESISTOR0603  [0603-RES]
R113  100K  RESISTOR0402-RES  [0402-RES]
R115  100K  RESISTOR0402-RES  [0402-RES]
R116  100K  RESISTOR0402-RES  [0402-RES]
R118  100K  RESISTOR0402-RES  [0402-RES]
R119  0, DNP  RESISTOR0603  [0603-RES]
R120  100K  RESISTOR0402-RES  [0402-RES]
R121  0, DNP  RESISTOR0603  [0603-RES]
R122  100K  RESISTOR0402-RES  [0402-RES]
R125  100K  RESISTOR0402-RES  [0402-RES]
R127  100K  RESISTOR0402-RES  [0402-RES]
R129  100K  RESISTOR0402-RES  [0402-RES]
R131  100K  RESISTOR0402-RES  [0402-RES]
R135  100K  RESISTOR0402-RES  [0402-RES]
R140  100K  RESISTOR0402-RES  [0402-RES]
R143  100K  RESISTOR0402-RES  [0402-RES]
R149  0  RESISTOR0402-RES  [0402-RES]
R150  0  RESISTOR0402-RES  [0402-RES]
R156  33  RESISTOR0402-RES  [0402-RES]
U3  TPD4S012DRY  TPD4S012DRYR  [SON-6(TI)-DRY]
U4  TPD4S012DRY  TPD4S012DRYR  [SON-6(TI)-DRY]
U8  TPS2105_DBV_5  [DBV5]
X3  USB1  USB_HOST_W/CHASSIS_GND  [USB_HOST_HORIZONTAL_W/CHASSIS_GND]
X4  10118192-0001LF  [10118192-0001LF(MICRO-USB-B-AMPHENOL-FCI)]

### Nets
3.3V: R109.1 R116.2 R118.2 R120.2 R122.2 R140.2 ; also sheet 1,2,5
5.0V [power]: C63.1 R95.2 R119.2 U8.1(EN) U8.5(IN1) ; also sheet 1,2
AIN0: SIP.B6(C:AIN0) ; also sheet 1
AIN1: SIP.C7(C:AIN1) ; also sheet 1
AIN2: SIP.B7(C:AIN2) ; also sheet 1
AIN3: SIP.A7(C:AIN3) ; also sheet 1
BATT_LED_2: R143.2 SIP.T5(C:LCD_DATA15_T5) ; also sheet 1
BT_EN: SIP.K17(C:K17) ; also sheet 5
CGND: X3.5(CG1) X3.6(CG2) X4.CGND1(SGND1) X4.CGND2(SGND2) X4.CGND3(SGND3) X4.CGND4(SGND4) X4.CGND5(SGND5) X4.CGND6(SGND6) ; also sheet 1,2,4
DCAN1_SILENT: SIP.M16(C:M16) ; also sheet 2
EQEP_1A: R16.2 SIP.V2(C:LCD_DATA12_V2) ; also sheet 1
EQEP_1B: R17.2 SIP.V3(C:LCD_DATA13_V3) ; also sheet 1
GND [ground]: C45.2 C46.2 C54.2 C55.2 C61.1 C62.2 C63.2 L4.1 R16.1 R17.1 R95.1 R110.2 R113.1 R115.1 R125.1 R127.1 R129.1 R131.1 R135.1 R143.1 R150.2 U3.4(GND) U4.4(GND) U8.2(GND) X4.GND ; also sheet 1,2,4,5
GNDA_ADC: C42.2 C43.2 C44.2 SIP.A6(C:VSSA_ADC_0) SIP.A9(C:VSSA_ADC_1) SIP.E8(C:VSSA_ADC_2)
GPIO1_25: SIP.U16(C:HDMIINT_GPIO1_25_U16) ; also sheet 1
GPIO3_1: SIP.H17(C:H17) ; also sheet 1
GPIO3_2: SIP.J15(C:J15) ; also sheet 1
MCASP0_AXR0: SIP.T16(C:USB1OC_GPIO1_26_T16) ; also sheet 5
MCASP0_AXR1: SIP.V17(C:HDMIDIS_GPIO1_27_V17) ; also sheet 5
MDIR_2B: R140.1 SIP.V4(C:LCD_DATA14_V4) ; also sheet 1
MDIR_3A: R118.1 SIP.R4(C:LCD_DATA3_R4) ; also sheet 1
MDIR_3B: R77.1 R116.1 SIP.R3(C:LCD_DATA2_R3) ; also sheet 1
MDIR_4A: R113.2 SIP.R1(C:LCD_DATA0_R1) ; also sheet 1
MDIR_4B: R115.2 SIP.R2(C:LCD_DATA1_R2) ; also sheet 1
MMC2_CLK: R76.1 ; also sheet 5
MMC2_CMD: SIP.J16(C:J16) ; also sheet 5
MMC2_DAT0: SIP.J17(C:J17) ; also sheet 5
MMC2_DAT1: SIP.J18(C:J18) ; also sheet 5
MMC2_DAT2: SIP.K15(C:K15) ; also sheet 5
MMC2_DAT3: SIP.H16(C:H16) ; also sheet 5
N$45: R76.2 SIP.L15(C:L15)
N$86: R135.2 SIP.U4(C:LCD_DATA11_U4)
N$110: C42.1 C43.1 R111.2 SIP.B9(C:ADC_VREFP)
N$115: R109.2 R110.1 SIP.C9(C:AIN7)
N$121: R149.1 SIP.P15(C:USB0_VBUS)
N$126: R150.1 SIP.P17(C:USB1_ID)
N$128 [power]: L4.2 X3.4(GND)
N$129: R156.1 SIP.T18(C:USB1_VBUS)
N$130 [power]: L5.2 X3.1(VBUS)
SD_BOOT: R77.2 ; also sheet 1
SERVO_EN: SIP.U3(C:LCD_DATA10_U3) ; also sheet 1
SPI1_SS1: SIP.H18(C:H18) ; also sheet 1
SVO1: SIP.U5(C:LCD_VSYNC_U5) ; also sheet 1
SVO2: SIP.V5(C:LCD_PCLK_V5) ; also sheet 1
SVO3: SIP.R5(C:LCD_HSYNC_R5) ; also sheet 1
SVO4: SIP.R6(C:LCD_DE_R6) ; also sheet 1
SVO5: R125.2 SIP.T3(C:LCD_DATA6_T3) ; also sheet 1
SVO6: R127.2 SIP.T4(C:LCD_DATA7_T4) ; also sheet 1
SVO7: R120.1 SIP.T1(C:LCD_DATA4_T1) ; also sheet 1
SVO8: R122.1 SIP.T2(C:LCD_DATA5_T2) ; also sheet 1
SYS_5V [power]: C62.1 R121.2 U8.3(IN2) ; also sheet 2
UART3_CTSN: SIP.M17(C:M17) ; also sheet 5
UART3_RTSN: SIP.M18(C:M18) ; also sheet 5
UART3_RX: SIP.L17(C:L17) ; also sheet 5
UART3_TX: SIP.L16(C:L16) ; also sheet 5
UART5_RX: R131.2 SIP.U2(C:LCD_DATA9_U2) ; also sheet 1
UART5_TX: R129.2 SIP.U1(C:LCD_DATA8_U1) ; also sheet 1
USB0_D_N: SIP.N18(C:USB0_DM) U3.2(D-) X4.D-
USB0_D_P: SIP.N17(C:USB0_DP) U3.1(D+) X4.D+
USB0_ID: SIP.P16(C:USB0_ID) U3.3(ID) X4.ID
USB0_VBUS: C54.1 R112.2 R149.2 U3.6(VBUS) X4.VBUS
USB1_D_N: SIP.R18(C:USB1_DM) U4.2(D-) X3.2(D-)
USB1_D_P: SIP.R17(C:USB1_DP) U4.1(D+) X3.3(D+)
USB1_VBUS: C45.1 C46.1 C55.1 C61.2 L5.1 R119.1 R121.1 R156.2 U4.6(VBUS) U8.4(OUT)
USB_DC [power]: R112.1 ; also sheet 2
V_DIV_BAT: SIP.A8(C:AIN6) ; also sheet 1
V_DIV_DC: SIP.B8(C:AIN5) ; also sheet 1
VDD_ADC: C44.1 R111.1 SIP.A4(C:VOUT_ADC_1P8V_0) SIP.A5(C:VOUT_ADC_1P8V_1) ; also sheet 1,4
WL_BT_OE: SIP.L18(C:L18) ; also sheet 5
WL_EN: SIP.K18(C:K18) ; also sheet 5
WLAN_IRQ: SIP.K16(C:K16) ; also sheet 5
Unconnected: SIP.C8(C:AIN4) SIP.F15(C:USB1_DRVVBUS) SIP.F16(C:USB0_DRVVBUS) SIP.M15(C:USB0_CE) SIP.P18(C:USB1_CE) U3.5(NC) U4.3(ID) U4.5(NC)

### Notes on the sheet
- Pulled down on Pg 1
- GPIO3_9
- GPIO0_28
- GPIO0_21
- GPIO3_10

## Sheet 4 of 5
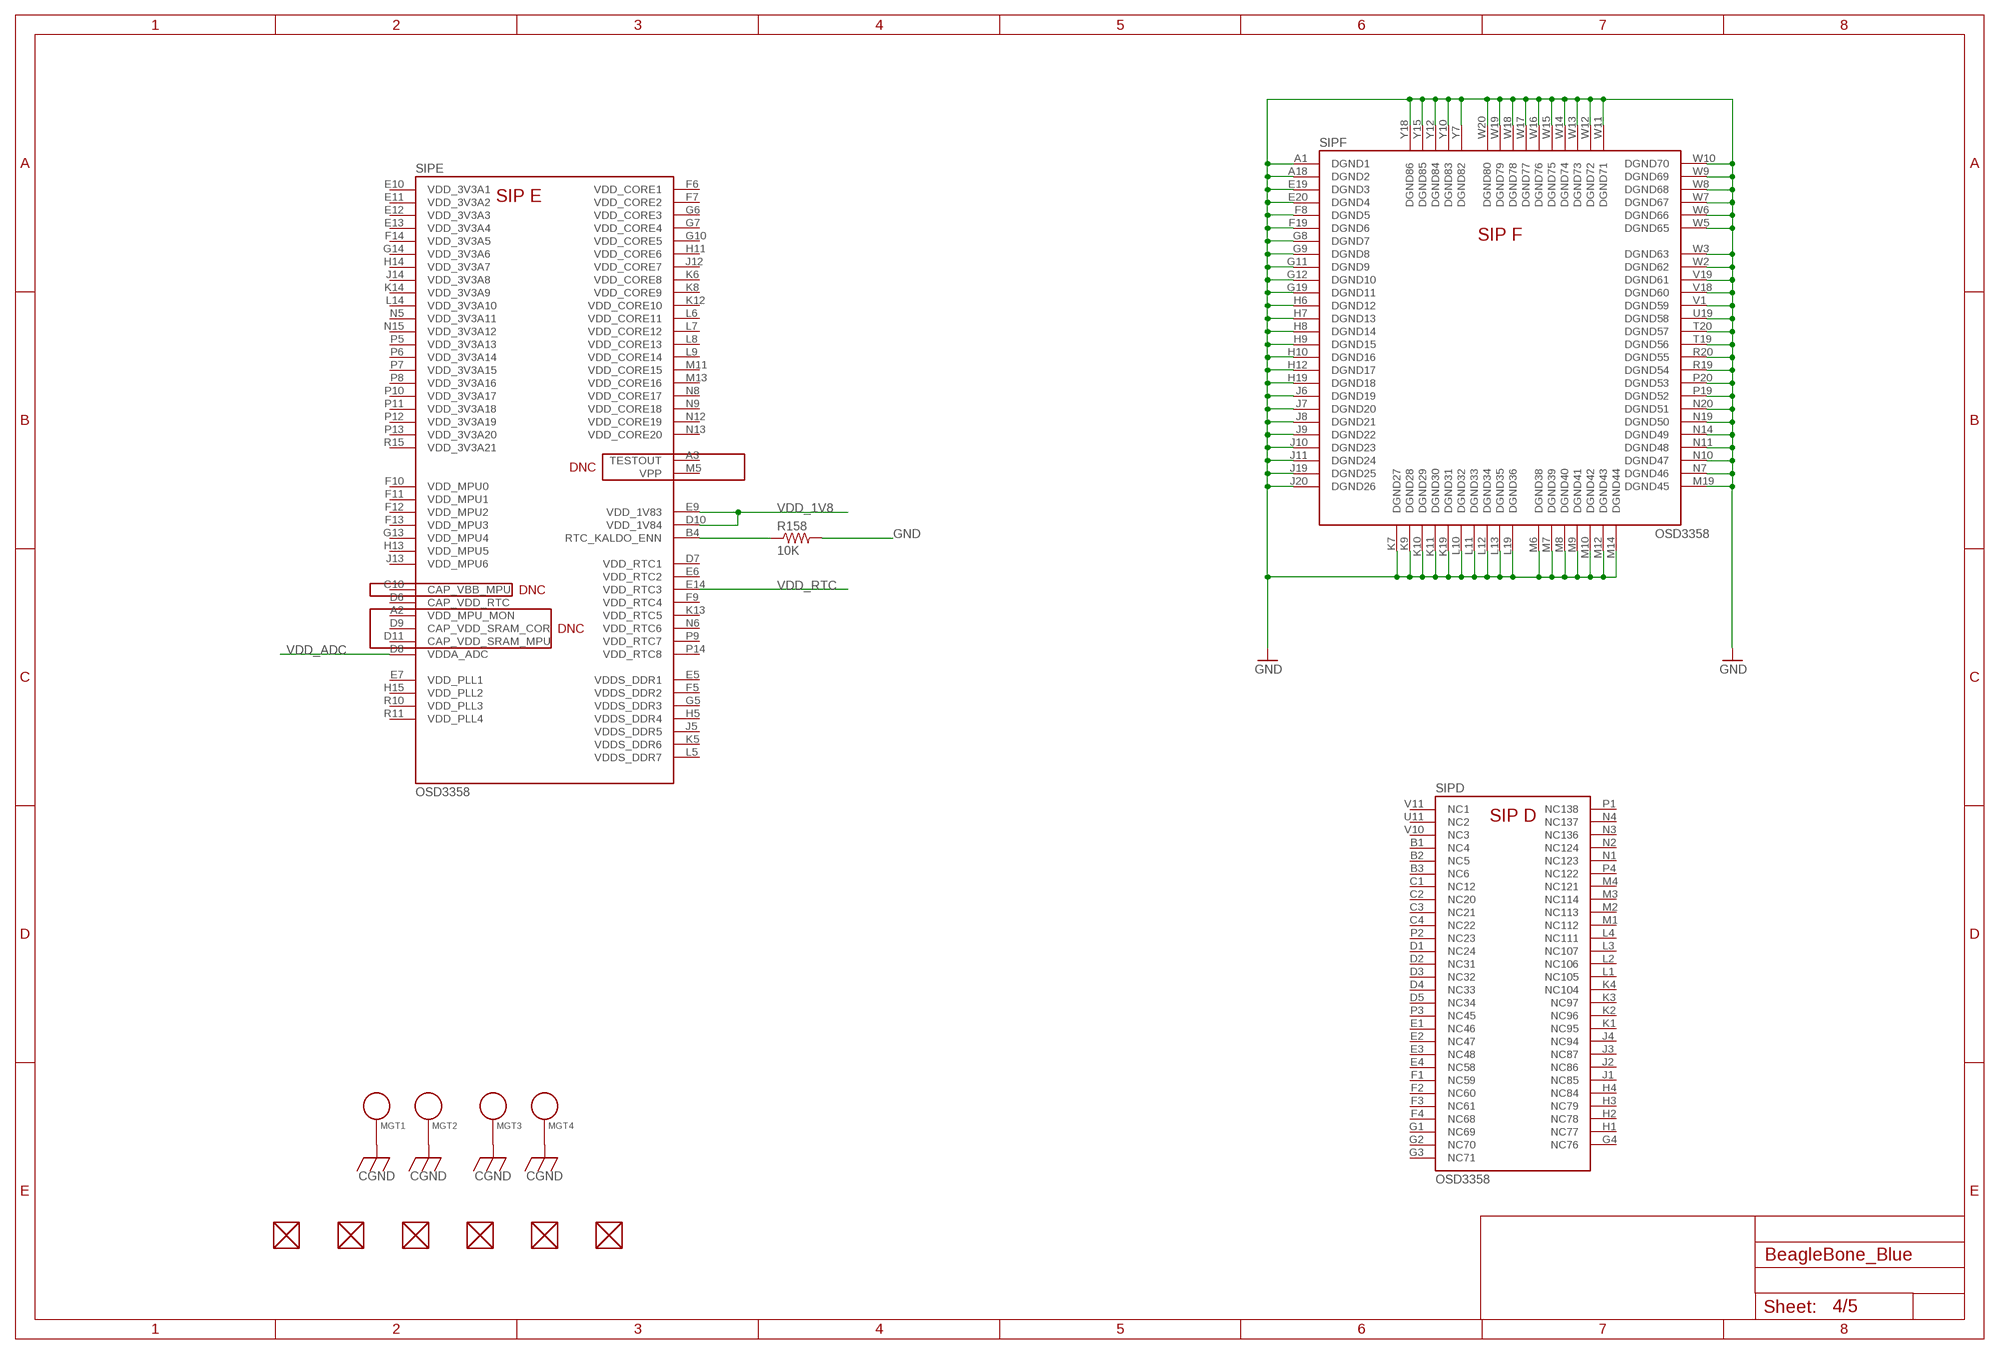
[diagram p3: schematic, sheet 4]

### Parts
FUD1  FIDUCIAL  [FIDUCIAL_40MIL]
FUD2  FIDUCIAL  [FIDUCIAL_40MIL]
FUD3  FIDUCIAL  [FIDUCIAL_40MIL]
FUD4  FIDUCIAL  [FIDUCIAL_40MIL]
FUD5  FIDUCIAL  [FIDUCIAL_40MIL]
FUD6  FIDUCIAL  [FIDUCIAL_40MIL]
MGT1  MOUNTING_HOLE  [MOUNTING_HOLE]
MGT2  MOUNTING_HOLE  [MOUNTING_HOLE]
MGT3  MOUNTING_HOLE  [MOUNTING_HOLE]
MGT4  MOUNTING_HOLE  [MOUNTING_HOLE]
R158  10K  RESISTOR0402-RES  [0402-RES]

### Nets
CGND: MGT1.P$1 MGT2.P$1 MGT3.P$1 MGT4.P$1 ; also sheet 1,2,3
GND [ground]: R158.2 SIP.A1(F:DGND1) SIP.A18(F:DGND2) SIP.E19(F:DGND3) SIP.E20(F:DGND4) SIP.F8(F:DGND5) SIP.F19(F:DGND6) SIP.G8(F:DGND7) SIP.G9(F:DGND8) SIP.G11(F:DGND9) SIP.G12(F:DGND10) SIP.G19(F:DGND11) SIP.H6(F:DGND12) SIP.H7(F:DGND13) SIP.H8(F:DGND14) SIP.H9(F:DGND15) SIP.H10(F:DGND16) SIP.H12(F:DGND17) SIP.H19(F:DGND18) SIP.J6(F:DGND19) SIP.J7(F:DGND20) SIP.J8(F:DGND21) SIP.J9(F:DGND22) SIP.J10(F:DGND23) SIP.J11(F:DGND24) SIP.J19(F:DGND25) SIP.J20(F:DGND26) SIP.K7(F:DGND27) SIP.K9(F:DGND28) SIP.K10(F:DGND29) SIP.K11(F:DGND30) SIP.K19(F:DGND31) SIP.L10(F:DGND32) SIP.L11(F:DGND33) SIP.L12(F:DGND34) SIP.L13(F:DGND35) SIP.L19(F:DGND36) SIP.M6(F:DGND38) SIP.M7(F:DGND39) SIP.M8(F:DGND40) SIP.M9(F:DGND41) SIP.M10(F:DGND42) SIP.M12(F:DGND43) SIP.M14(F:DGND44) SIP.M19(F:DGND45) SIP.N7(F:DGND46) SIP.N10(F:DGND47) SIP.N11(F:DGND48) SIP.N14(F:DGND49) SIP.N19(F:DGND50) SIP.N20(F:DGND51) SIP.P19(F:DGND52) SIP.P20(F:DGND53) SIP.R19(F:DGND54) SIP.R20(F:DGND55) SIP.T19(F:DGND56) SIP.T20(F:DGND57) SIP.U19(F:DGND58) SIP.V1(F:DGND59) SIP.V18(F:DGND60) SIP.V19(F:DGND61) SIP.W2(F:DGND62) SIP.W3(F:DGND63) SIP.W5(F:DGND65) SIP.W6(F:DGND66) SIP.W7(F:DGND67) SIP.W8(F:DGND68) SIP.W9(F:DGND69) SIP.W10(F:DGND70) SIP.W11(F:DGND71) SIP.W12(F:DGND72) SIP.W13(F:DGND73) SIP.W14(F:DGND74) SIP.W15(F:DGND75) SIP.W16(F:DGND76) SIP.W17(F:DGND77) SIP.W18(F:DGND78) SIP.W19(F:DGND79) SIP.W20(F:DGND80) SIP.Y7(F:DGND82) SIP.Y10(F:DGND83) SIP.Y12(F:DGND84) SIP.Y15(F:DGND85) SIP.Y18(F:DGND86) ; also sheet 1,2,3,5
N$131: R158.1 SIP.B4(E:RTC_KALDO_ENN)
VDD_1V8: SIP.D10(E:VDD_1V84) SIP.E9(E:VDD_1V83) ; also sheet 2,5
VDD_ADC: SIP.D8(E:VDDA_ADC) ; also sheet 1,3
VDD_RTC: SIP.E14(E:VDD_RTC3) ; also sheet 2
Unconnected: FUD1.P$1 FUD2.P$1 FUD3.P$1 FUD4.P$1 FUD5.P$1 FUD6.P$1 SIP.A2(E:VDD_MPU_MON) SIP.A3(E:TESTOUT) SIP.B1(D:NC4) SIP.B2(D:NC5) SIP.B3(D:NC6) SIP.C1(D:NC12) SIP.C2(D:NC20) SIP.C3(D:NC21) SIP.C4(D:NC22) SIP.C10(E:CAP_VBB_MPU) SIP.D1(D:NC24) SIP.D2(D:NC31) SIP.D3(D:NC32) SIP.D4(D:NC33) SIP.D5(D:NC34) SIP.D6(E:CAP_VDD_RTC) SIP.D7(E:VDD_RTC1) SIP.D9(E:CAP_VDD_SRAM_COR) SIP.D11(E:CAP_VDD_SRAM_MPU) SIP.E1(D:NC46) SIP.E2(D:NC47) SIP.E3(D:NC48) SIP.E4(D:NC58) SIP.E5(E:VDDS_DDR1) SIP.E6(E:VDD_RTC2) SIP.E7(E:VDD_PLL1) SIP.E10(E:VDD_3V3A1) SIP.E11(E:VDD_3V3A2) SIP.E12(E:VDD_3V3A3) SIP.E13(E:VDD_3V3A4) SIP.F1(D:NC59) SIP.F2(D:NC60) SIP.F3(D:NC61) SIP.F4(D:NC68) SIP.F5(E:VDDS_DDR2) SIP.F6(E:VDD_CORE1) SIP.F7(E:VDD_CORE2) SIP.F9(E:VDD_RTC4) SIP.F10(E:VDD_MPU0) SIP.F11(E:VDD_MPU1) SIP.F12(E:VDD_MPU2) SIP.F13(E:VDD_MPU3) SIP.F14(E:VDD_3V3A5) SIP.G1(D:NC69) SIP.G2(D:NC70) SIP.G3(D:NC71) SIP.G4(D:NC76) SIP.G5(E:VDDS_DDR3) SIP.G6(E:VDD_CORE3) SIP.G7(E:VDD_CORE4) SIP.G10(E:VDD_CORE5) SIP.G13(E:VDD_MPU4) SIP.G14(E:VDD_3V3A6) SIP.H1(D:NC77) SIP.H2(D:NC78) SIP.H3(D:NC79) SIP.H4(D:NC84) SIP.H5(E:VDDS_DDR4) SIP.H11(E:VDD_CORE6) SIP.H13(E:VDD_MPU5) SIP.H14(E:VDD_3V3A7) SIP.H15(E:VDD_PLL2) SIP.J1(D:NC85) SIP.J2(D:NC86) SIP.J3(D:NC87) SIP.J4(D:NC94) SIP.J5(E:VDDS_DDR5) SIP.J12(E:VDD_CORE7) SIP.J13(E:VDD_MPU6) SIP.J14(E:VDD_3V3A8) SIP.K1(D:NC95) SIP.K2(D:NC96) SIP.K3(D:NC97) SIP.K4(D:NC104) SIP.K5(E:VDDS_DDR6) SIP.K6(E:VDD_CORE8) SIP.K8(E:VDD_CORE9) SIP.K12(E:VDD_CORE10) SIP.K13(E:VDD_RTC5) SIP.K14(E:VDD_3V3A9) SIP.L1(D:NC105) SIP.L2(D:NC106) SIP.L3(D:NC107) SIP.L4(D:NC111) SIP.L5(E:VDDS_DDR7) SIP.L6(E:VDD_CORE11) SIP.L7(E:VDD_CORE12) SIP.L8(E:VDD_CORE13) SIP.L9(E:VDD_CORE14) SIP.L14(E:VDD_3V3A10) SIP.M1(D:NC112) SIP.M2(D:NC113) SIP.M3(D:NC114) SIP.M4(D:NC121) SIP.M5(E:VPP) SIP.M11(E:VDD_CORE15) SIP.M13(E:VDD_CORE16) SIP.N1(D:NC123) SIP.N2(D:NC124) SIP.N3(D:NC136) SIP.N4(D:NC137) SIP.N5(E:VDD_3V3A11) SIP.N6(E:VDD_RTC6) SIP.N8(E:VDD_CORE17) SIP.N9(E:VDD_CORE18) SIP.N12(E:VDD_CORE19) SIP.N13(E:VDD_CORE20) SIP.N15(E:VDD_3V3A12) SIP.P1(D:NC138) SIP.P2(D:NC23) SIP.P3(D:NC45) SIP.P4(D:NC122) SIP.P5(E:VDD_3V3A13) SIP.P6(E:VDD_3V3A14) SIP.P7(E:VDD_3V3A15) SIP.P8(E:VDD_3V3A16) SIP.P9(E:VDD_RTC7) SIP.P10(E:VDD_3V3A17) SIP.P11(E:VDD_3V3A18) SIP.P12(E:VDD_3V3A19) SIP.P13(E:VDD_3V3A20) SIP.P14(E:VDD_RTC8) SIP.R10(E:VDD_PLL3) SIP.R11(E:VDD_PLL4) SIP.R15(E:VDD_3V3A21) SIP.U11(D:NC2) SIP.V10(D:NC3) SIP.V11(D:NC1)

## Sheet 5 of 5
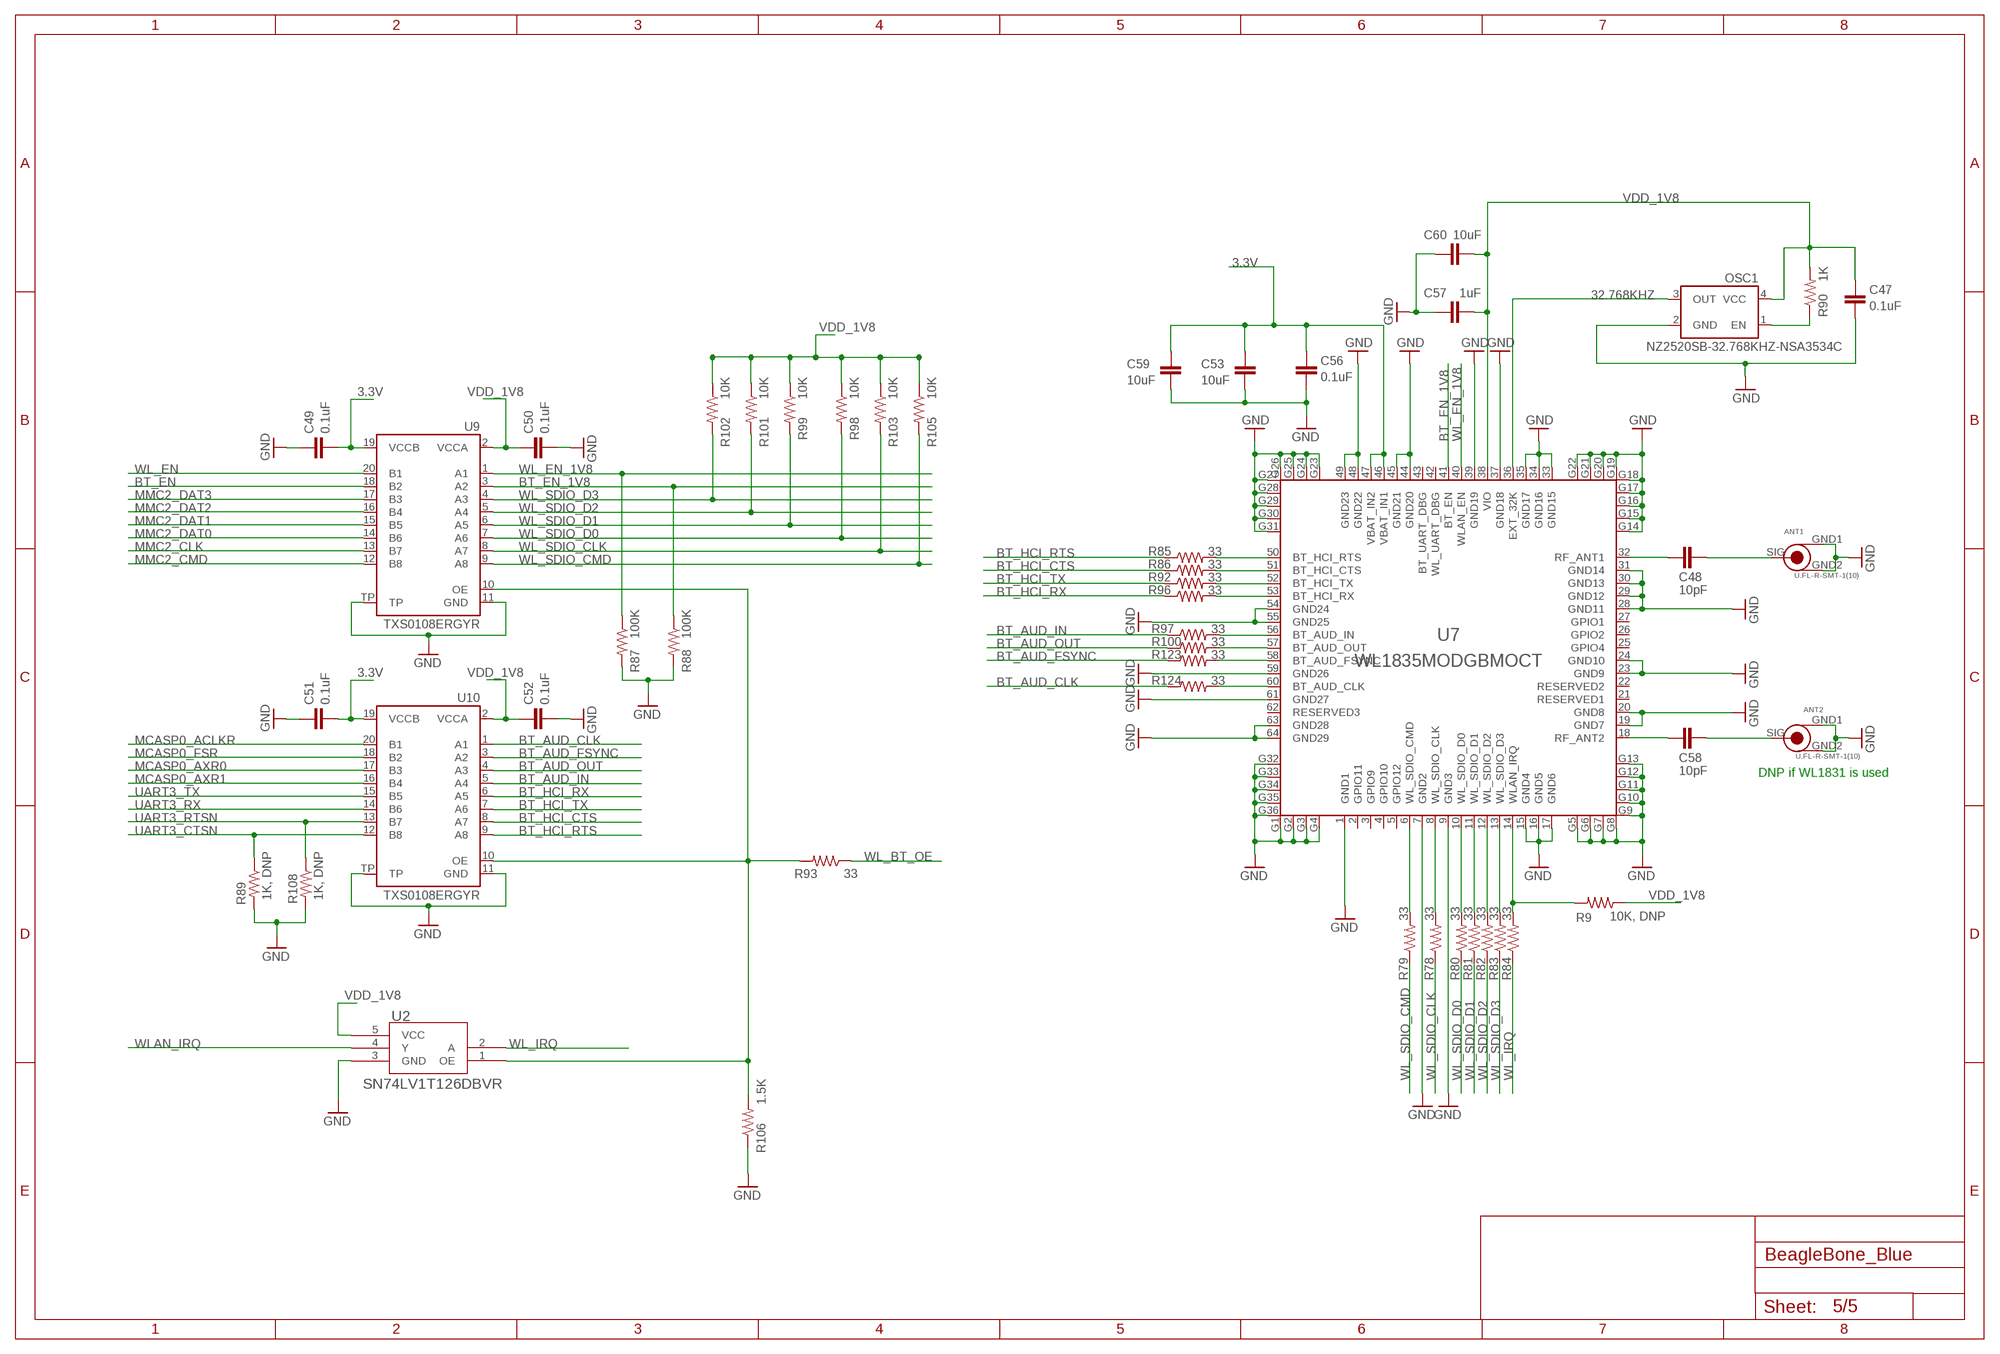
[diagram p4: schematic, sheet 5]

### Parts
ANT1  U.FL-R-SMT-1(10)  U.FL-R-SMT-1  [U.FL-R-SMT-1]
ANT2  U.FL-R-SMT-1(10)  U.FL-R-SMT-1  [U.FL-R-SMT-1]
C47  0.1uF  CAP0402-CAP  [0402-CAP]
C48  10pF  CAP0402-CAP  [0402-CAP]
C49  0.1uF  CAP0402-CAP  [0402-CAP]
C50  0.1uF  CAP0402-CAP  [0402-CAP]
C51  0.1uF  CAP0402-CAP  [0402-CAP]
C52  0.1uF  CAP0402-CAP  [0402-CAP]
C53  10uF  CAP0805  [0805]
C56  0.1uF  CAP0402-CAP  [0402-CAP]
C57  1uF  CAP0402-CAP  [0402-CAP]
C58  10pF  CAP0402-CAP  [0402-CAP]
C59  10uF  CAP0805  [0805]
C60  10uF  CAP0805  [0805]
OSC1  NZ2520SB-32.768KHZ-NSA3534C  OSCILLATOR  [NZ2520S]
R9  10K, DNP  RESISTOR0402-RES  [0402-RES]
R78  33  RESISTOR0402-RES  [0402-RES]
R79  33  RESISTOR0402-RES  [0402-RES]
R80  33  RESISTOR0402-RES  [0402-RES]
R81  33  RESISTOR0402-RES  [0402-RES]
R82  33  RESISTOR0402-RES  [0402-RES]
R83  33  RESISTOR0402-RES  [0402-RES]
R84  33  RESISTOR0402-RES  [0402-RES]
R85  33  RESISTOR0402-RES  [0402-RES]
R86  33  RESISTOR0402-RES  [0402-RES]
R87  100K  RESISTOR0402-RES  [0402-RES]
R88  100K  RESISTOR0402-RES  [0402-RES]
R89  1K, DNP  RESISTOR0402-RES  [0402-RES]
R90  1K  RESISTOR0402-RES  [0402-RES]
R92  33  RESISTOR0402-RES  [0402-RES]
R93  33  RESISTOR0402-RES  [0402-RES]
R96  33  RESISTOR0402-RES  [0402-RES]
R97  33  RESISTOR0402-RES  [0402-RES]
R98  10K  RESISTOR0402-RES  [0402-RES]
R99  10K  RESISTOR0402-RES  [0402-RES]
R100  33  RESISTOR0402-RES  [0402-RES]
R101  10K  RESISTOR0402-RES  [0402-RES]
R102  10K  RESISTOR0402-RES  [0402-RES]
R103  10K  RESISTOR0402-RES  [0402-RES]
R105  10K  RESISTOR0402-RES  [0402-RES]
R106  1.5K  RESISTOR0402-RES  [0402-RES]
R108  1K, DNP  RESISTOR0402-RES  [0402-RES]
R123  33  RESISTOR0402-RES  [0402-RES]
R124  33  RESISTOR0402-RES  [0402-RES]
U2  SN74LV1T126DBVR  [BEAGLEBONE_BLUE_SOT23-5]
U7  WL1835MODGBMOCT  WL1835MOD  [MOC-100(TI)]
U9  TXS0108ERGYR  [R-PVQFN-N20(TI)]
U10  TXS0108ERGYR  [R-PVQFN-N20(TI)]

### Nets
3.3V: C49.2 C51.2 C53.1 C56.1 C59.1 U7.46(VBAT_IN1) U7.47(VBAT_IN2) U9.19(VCCB) U10.19(VCCB) ; also sheet 1,2,3
32.768KHZ: OSC1.3(OUT) U7.36(EXT_32K)
ALT.BUFF.OE: R93.2 R106.2 U2.1(OE) U9.10(OE) U10.10(OE)
ANT1_A: C48.2 U7.32(RF_ANT1)
ANT1_B: ANT1.SIG C48.1
ANT2_A: C58.2 U7.18(RF_ANT2)
ANT2_B: ANT2.SIG C58.1
BT_AUD_CLK: R124.1 U10.1(A1)
BT_AUD_FSYNC: R123.1 U10.3(A2)
BT_AUD_IN: R97.1 U10.5(A4)
BT_AUD_OUT: R100.1 U10.4(A3)
BT_EN: U9.18(B2) ; also sheet 3
BT_EN_1V8: R88.1 U7.41(BT_EN) U9.3(A2)
BT_HCI_CTS: R86.1 U10.8(A7)
BT_HCI_RTS: R85.1 U10.9(A8)
BT_HCI_RX: R96.1 U10.6(A5)
BT_HCI_TX: R92.1 U10.7(A6)
GND [ground]: ANT1.GND1 ANT1.GND2 ANT2.GND1 ANT2.GND2 C47.2 C49.1 C50.2 C51.1 C52.2 C53.2 C56.2 C57.1 C59.2 C60.1 OSC1.2(GND) R87.2 R88.2 R89.2 R106.1 R108.2 U2.3(GND) U7.1(GND1) U7.7(GND2) U7.9(GND3) U7.15(GND4) U7.16(GND5) U7.17(GND6) U7.19(GND7) U7.20(GND8) U7.23(GND9) U7.24(GND10) U7.28(GND11) U7.29(GND12) U7.30(GND13) U7.31(GND14) U7.33(GND15) U7.34(GND16) U7.35(GND17) U7.37(GND18) U7.39(GND19) U7.44(GND20) U7.45(GND21) U7.48(GND22) U7.49(GND23) U7.54(GND24) U7.55(GND25) U7.59(GND26) U7.61(GND27) U7.63(GND28) U7.64(GND29) U7.G1 U7.G2 U7.G3 U7.G4 U7.G5 U7.G6 U7.G7 U7.G8 U7.G9 U7.G10 U7.G11 U7.G12 U7.G13 U7.G14 U7.G15 U7.G16 U7.G17 U7.G18 U7.G19 U7.G20 U7.G21 U7.G22 U7.G23 U7.G24 U7.G25 U7.G26 U7.G27 U7.G28 U7.G29 U7.G30 U7.G31 U7.G32 U7.G33 U7.G34 U7.G35 U7.G36 U9.11(GND) U9.TP U10.11(GND) U10.TP ; also sheet 1,2,3,4
MCASP0_ACLKR: U10.20(B1) ; also sheet 2
MCASP0_AXR0: U10.17(B3) ; also sheet 3
MCASP0_AXR1: U10.16(B4) ; also sheet 3
MCASP0_FSR: U10.18(B2) ; also sheet 2
MMC2_CLK: U9.13(B7) ; also sheet 3
MMC2_CMD: U9.12(B8) ; also sheet 3
MMC2_DAT0: U9.14(B6) ; also sheet 3
MMC2_DAT1: U9.15(B5) ; also sheet 3
MMC2_DAT2: U9.16(B4) ; also sheet 3
MMC2_DAT3: U9.17(B3) ; also sheet 3
N$7: OSC1.1(EN) R90.1
N$43: R100.2 U7.57(BT_AUD_OUT)
N$103: R9.2 R84.2 U7.14(WLAN_IRQ)
N$104: R83.2 U7.13(WL_SDIO_D3)
N$105: R82.2 U7.12(WL_SDIO_D2)
N$106: R81.2 U7.11(WL_SDIO_D1)
N$107: R80.2 U7.10(WL_SDIO_D0)
N$108: R78.2 U7.8(WL_SDIO_CLK)
N$111: R79.2 U7.6(WL_SDIO_CMD)
N$112: R85.2 U7.50(BT_HCI_RTS)
N$113: R86.2 U7.51(BT_HCI_CTS)
N$114: R92.2 U7.52(BT_HCI_TX)
N$116: R96.2 U7.53(BT_HCI_RX)
N$146: R97.2 U7.56(BT_AUD_IN)
N$148: R123.2 U7.58(BT_AUD_FSYNC)
N$149: R124.2 U7.60(BT_AUD_CLK)
UART3_CTSN: R89.1 U10.12(B8) ; also sheet 3
UART3_RTSN: R108.1 U10.13(B7) ; also sheet 3
UART3_RX: U10.14(B6) ; also sheet 3
UART3_TX: U10.15(B5) ; also sheet 3
VDD_1V8: C47.1 C50.1 C52.1 C57.2 C60.2 OSC1.4(VCC) R9.1 R90.2 R98.1 R99.1 R101.1 R102.1 R103.1 R105.1 U2.5(VCC) U7.38(VIO) U9.2(VCCA) U10.2(VCCA) ; also sheet 2,4
WL_BT_OE: R93.1 ; also sheet 3
WL_EN: U9.20(B1) ; also sheet 3
WL_EN_1V8: R87.1 U7.40(WLAN_EN) U9.1(A1)
WL_IRQ: R84.1 U2.2(A)
WL_SDIO_CLK: R78.1 R103.2 U9.8(A7)
WL_SDIO_CMD: R79.1 R105.2 U9.9(A8)
WL_SDIO_D0: R80.1 R98.2 U9.7(A6)
WL_SDIO_D1: R81.1 R99.2 U9.6(A5)
WL_SDIO_D2: R82.1 R101.2 U9.5(A4)
WL_SDIO_D3: R83.1 R102.2 U9.4(A3)
WLAN_IRQ: U2.4(Y) ; also sheet 3
Unconnected: U7.2(GPIO11) U7.3(GPIO9) U7.4(GPIO10) U7.5(GPIO12) U7.21(RESERVED1) U7.22(RESERVED2) U7.25(GPIO4) U7.26(GPIO2) U7.27(GPIO1) U7.42(WL_UART_DBG) U7.43(BT_UART_DBG) U7.62(RESERVED3)

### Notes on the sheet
- DNP if WL1831 is used

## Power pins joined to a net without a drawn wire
VIN_BAT_0: SIP.Y2(A:VIN_BAT_0)
VIN_BAT_1: SIP.Y3(A:VIN_BAT_1)

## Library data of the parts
0 1-3 G ON R WIFI = BeagleBone_Blue:LED: LEDs
5VREG = BeagleBone_Blue:AP1509: 150KHz, 2A PWM BUCK DC/DC CONVERTER
6VREG = Strawson_Eagle_Lib:AOZ1284
12V = GHI:PJ-102B_POWER_CON
ADC GP0 GP1 GPS S1.1 S1.2 = Strawson_Eagle_Lib:JST_SH_6
ANT1 ANT2 = GHI-Connectors:U.FL-R-SMT-1
B0 B1-B3 CHG = SparkFun-LED:LED: LEDs
BAL = Strawson_Eagle_Lib:BQ29209: BQ29209 2-CELL Balance and Overvoltage Protection
BMP = Strawson_Eagle_Lib:BMP280: BOSCH BMP280 Digital Pressure Sensor
C1 C2 C4 C6 C8-C10 C13-C15 C17-C19 C21 C22 C24 C27-C52 C54-C58 C61-C63 = Strawson_Eagle_Lib:CAP: Capacitor
C3 C5 C7 C12 C16 C20 C23 C25 C26 C53 C59 C60 = SparkFun-Capacitors:CAP: Capacitor
C11 = adafruit:CPOL-US: POLARIZED CAPACITOR, American symbol
CAN E1-E4 I2C PWR UT0 UT1 UT5 = Strawson_Eagle_Lib:JST_SH_4
CHGIC = Strawson_Eagle_Lib:MP2615
D1-D3 = BeagleBone_Blue:DIODE: Diode
D9 = Strawson_Eagle_Lib:DIODE: Diode
DSM2 = Strawson_Eagle_Lib:JST_ZH_3
EMU0 EMU1 TCK TDI TDO TMS TP1 TP12 TRSTN = testpad:TPSQ: Test pad
FUD1-FUD6 = GHI:FIDUCIAL
GND WP = BeagleBone_Blue:GHI2_TESTPAD/W_HOLE_1X1
H1 H2 = SparkFun:TB6612FNG: Toshiba 1A motor driver
IMU = Strawson_Eagle_Lib:MPU-9250: 314990005; MPN: MPU-9250
J2 = BeagleBone_Blue:STRAWSON_EAGLE_LIB_SERVO_HEADERS_8X
L1 L2 = SparkFun-Passives:INDUCTOR: Inductors; PROD_ID: NDUC-11627; VALUE: 33uH
L3 = Strawson_Eagle_Lib:INDUCTOR: Inductors; VALUE: 3.3uH
L4 L5 = Seeed-OPL-Inductor:INDUCTOR/FERRITE-BEAD
LIPO = Strawson_Eagle_Lib:JST_XH_3-PIN
M1-M4 = Strawson_Eagle_Lib:JST_ZH_2
MGT1-MGT4 = BeagleBoneBlack:MOUNTING_HOLE: Chassis Mounting Hole w/GND connection ability
MOD PAU POW RST SD = SparkFun-Electromechanical:SWITCH-MOMENTARY-2: Various NO switches- pushbuttons, reed, etc; PROD_ID: SWCH-00815
OSC1 = GHI-IC:OSCILLATOR
PROT = Strawson_Eagle_Lib:S-8261
Q1 = Strawson_Eagle_Lib:MOSFET-NCHANNEL: Common NMOSFET Parts MFG P/NStore IDProd ID FDD8780TRANS-09984 SI7820DNTRANS-11055 FDS6630AIC-08089 2N7002PWTRANS-11151 FQP30N06L COM-10213TRANS-10060 BSS123LT1GTRANS-08345 BSS138TRANS-00830 BS170 2N7000
R1-R3 R5-R103 R105 R106 R108-R111 R113 R115 R116 R118 R120 R122-R125 R127 R129 R131 R135 R140 R143 R149 R150 R156 R158 = Strawson_Eagle_Lib:RESISTOR: Resistor
R4 R104 R112 R119 R121 = SparkFun-Resistors:RESISTOR: Resistor
R107 = rcl:R-US_: RESISTOR, American symbol
SIP = BeagleBone_Blue:OSD3358: Octavo Systems LLC - OSD3358 Rev A
TP5 = BeagleBone_Blue:TP: Test pad
U1 = BeagleBone_Blue:TCAN1051HV; DATASHEETURL: http://www.ti.com/lit/ds/symlink/tcan1051hv.pdf; DESCRIPTION: CAN Transceiver; FAMILY_NAME: CAN Transceiver; GENERIC_PART_NUMBER: TCAN1051HV; INDUSTRY_STD_PKG_TYPE: SOIC; MANUFACTURER: Texas Instruments; MANUFACTURER_PART_NUMBER: TCAN1051HVD; PACKAGE_DESIGNATOR: D; PIN_COUNT: 8; VENDOR: Texas Instruments
U2 = BeagleBone_Blue:SN74LV1T126DBVR
U3 U4 = GHI-IC:TPD4S012DRYR
U5 = Microchip-24LCxxx:24LC_: IC, I2C Serial EEPROM,SOT-23-5; MPN: 24LC32AT-I/OT; OC_FARNELL: 1700993; OC_NEWARK: 08P0113; PACKAGE: SOT-23-5; SUPPLIER: MICROCHIP
U6 = BeagleBone_Blue:SN74LVC1G07_DCK_5; DATASHEETURL: http://www.ti.com/lit/gpn/SN74LVC1G07; DESCRIPTION: Single Buffer/Driver With Open-Drain Output; FAMILY_NAME: LL BUFFER AND DRIVER WITH OPEN-DRAIN OUTPUT; GENERIC_PART_NUMBER: SN74LVC1G07; INDUSTRY_STD_PKG_TYPE: SC70; MANUFACTURER: Texas Instruments; MANUFACTURER_PART_NUMBER: sn74lvc1g07_dck_5; PACKAGE_DESIGNATOR: DCK; PIN_COUNT: 5; VENDOR: Texas Instruments
U7 = GHI-IC:WL1835MOD
U8 = BeagleBone_Blue:TPS2105_DBV_5; DATASHEETURL: http://www.ti.com/lit/gpn/TPS2105; DESCRIPTION: 2.7-5.5V Dual In/Single Out MOSFET, 0.5A Main/0.1A Aux Input, Act-High Enable, Industrial Temp.; FAMILY_NAME: POWER MULTIPLEXER (MUX); GENERIC_PART_NUMBER: TPS2105; INDUSTRY_STD_PKG_TYPE: SOT-23; MANUFACTURER: Texas Instruments; MANUFACTURER_PART_NUMBER: tps2105_dbv_5; PACKAGE_DESIGNATOR: DBV; PIN_COUNT: 5; VENDOR: Texas Instruments
U9 U10 = GHI-IC:TXS0108ERGYR
U13 = GHI-IC:EMMC04G-S100-B08U
X2 = GHI-Connectors:SCHA5B0200(ALPS_USD)
X3 = GHI2:USB_HOST_W/CHASSIS_GND
X4 = GHI-Connectors:10118192-0001LF: Amphenol FCI Micro USB Type B Complete Surface Mount (SMT) no guide holes
Y1 = GHI2:CRYSTAL_5X3.2MM
Y2 = GHI2:CRYSTAL_3.2X1.5

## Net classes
0 default: width 0.152 mm, drill 0.254 mm, clearance 0.152 mm
1 ground: width 0.152 mm, drill 0.254 mm, clearance 0.152 mm
2 usb: width 0.152 mm, drill 0.254 mm, clearance 0.152 mm
3 power: width 0.152 mm, drill 0.254 mm, clearance 0.152 mm

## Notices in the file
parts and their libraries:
SparkFun-Aesthetics: Licensing: CC v3.0 Share-Alike You are welcome to use this library for commercial purposes.
